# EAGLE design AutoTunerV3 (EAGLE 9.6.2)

## Sheet 1 of 4: mcu
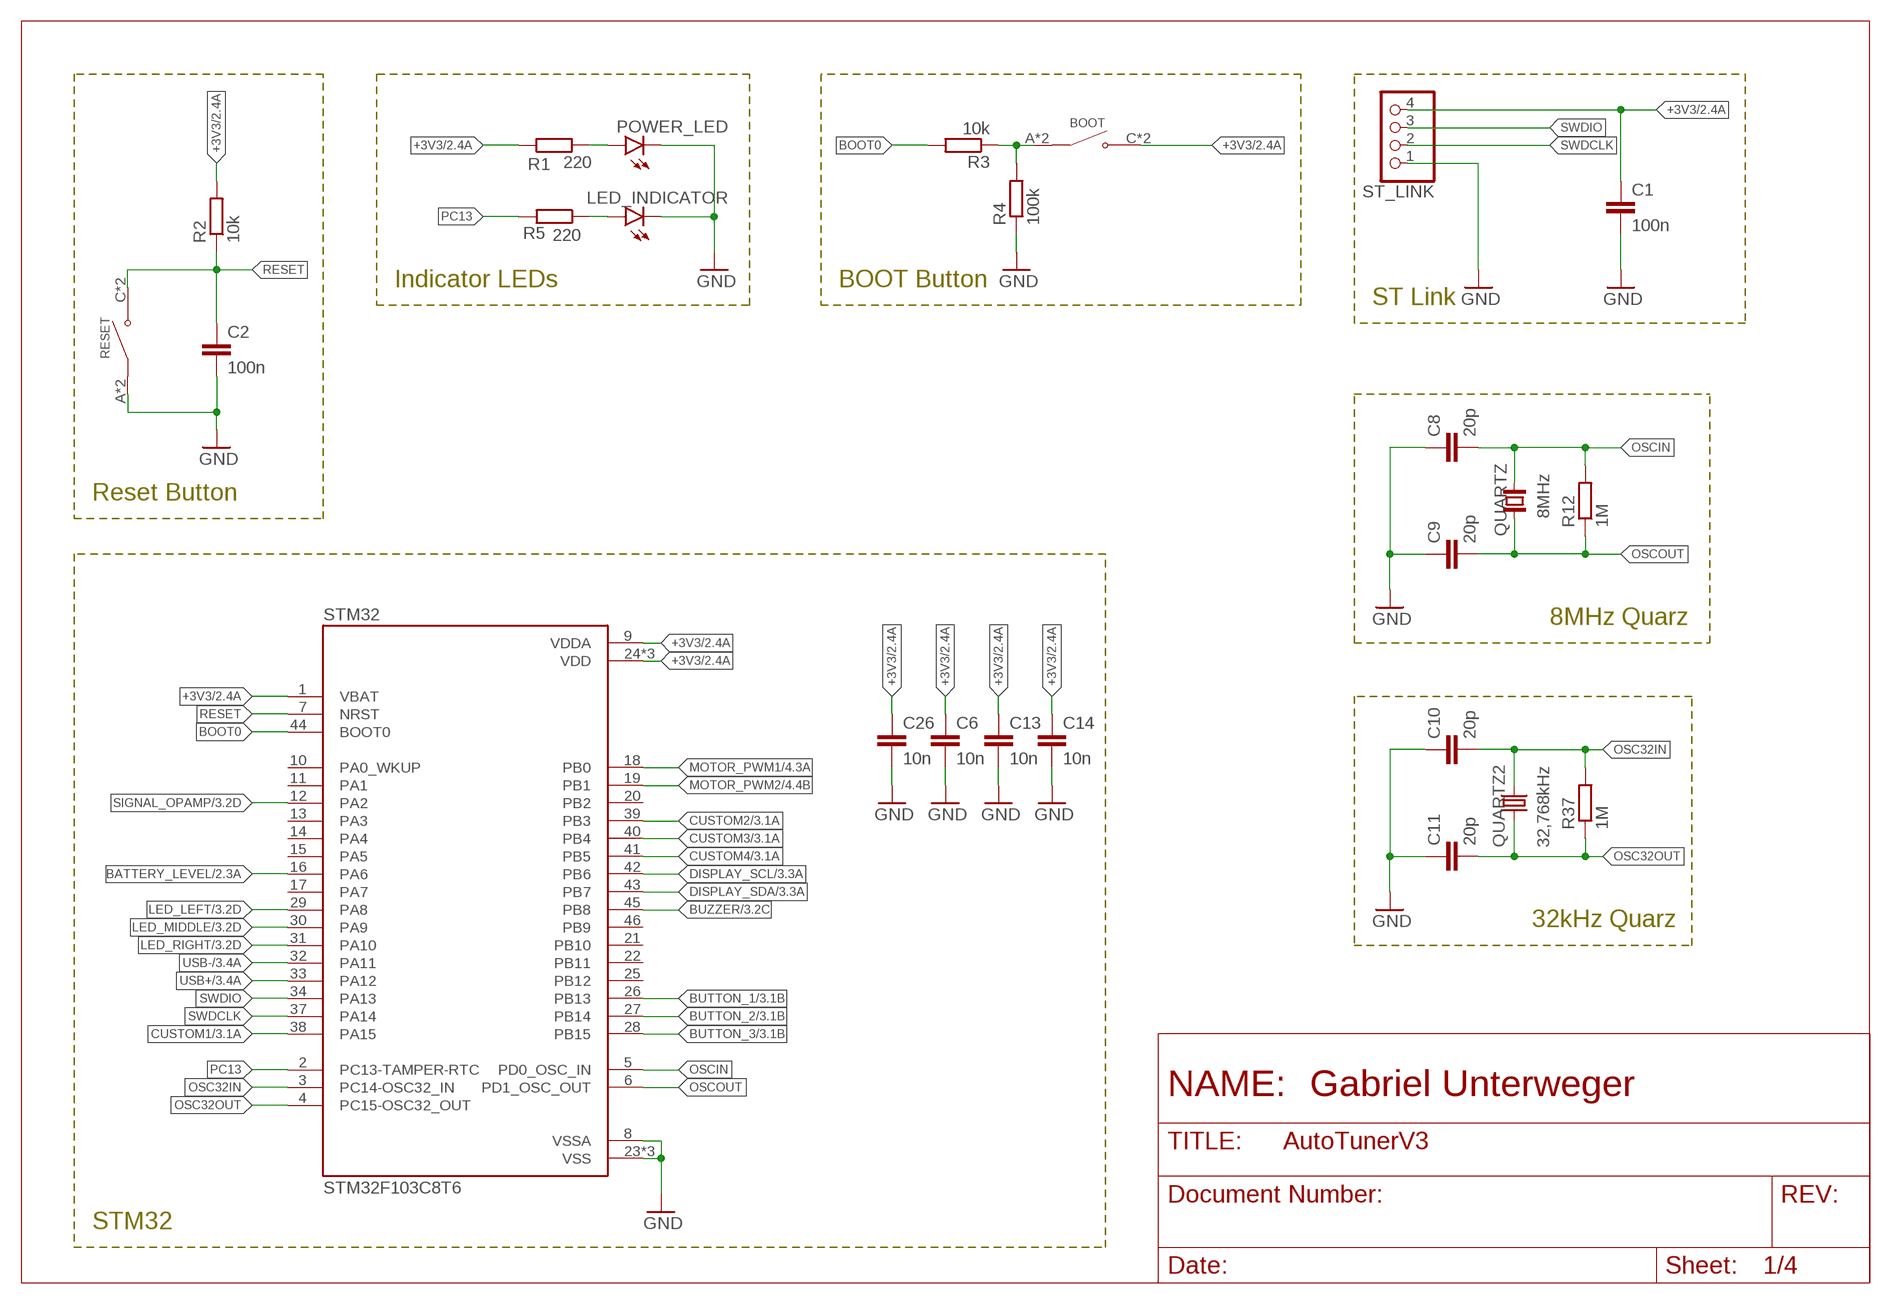
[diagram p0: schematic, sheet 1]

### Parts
BOOT  TS-1187A-B-A-B  [SW_TS-1187A-B-A-B]
C1  100n  C-EUC0805  [C0805]
C2  100n  C-EUC0805  [C0805]
C6  10n  C-EUC0805  [C0805]
C8  20p  C-EUC0805  [C0805]
C9  20p  C-EUC0805  [C0805]
C10  20p  C-EUC0805  [C0805]
C11  20p  C-EUC0805  [C0805]
C13  10n  C-EUC0805  [C0805]
C14  10n  C-EUC0805  [C0805]
C26  10n  C-EUC0805  [C0805]
LED_INDICATOR  LEDCHIPLED_0805  [CHIPLED_0805]
POWER_LED  LEDCHIPLED_0805  [CHIPLED_0805]
QUARTZ  8MHz  CRYSTAL_NX5032GA  [CRYSTAL_2-SMD-5X3]
QUARTZ2  32,768kHz  KX-327-NHF  [3.2X1.5]
R1  220  R-EU_R0805  [R0805]
R2  10k  R-EU_R0805  [R0805]
R3  10k  R-EU_R0805  [R0805]
R4  100k  R-EU_R0805  [R0805]
R5  220  R-EU_R0805  [R0805]
R12  1M  R-EU_R0805  [R0805]
R37  1M  R-EU_R0805  [R0805]
RESET  TS-1187A-B-A-B  [SW_TS-1187A-B-A-B]
ST_LINK  PINHD-1X4/90  [1X04/90]
STM32  STM32F103C8T6  [QFP50P900X900X160-48N]

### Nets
+3V3: BOOT.C(NO) BOOT.D(NO) C1.1 C6.1 C13.1 C14.1 C26.1 R1.1 R2.2 ST_LINK.4 STM32.1(VBAT) STM32.9(VDDA) STM32.24(VDD) STM32.36(VDD) STM32.48(VDD) ; also sheet 2,3,4
BATTERY_LEVEL: STM32.16(PA6) ; also sheet 2
BOOT0: R3.2 STM32.44(BOOT0)
BUTTON_1: STM32.26(PB13) ; also sheet 3
BUTTON_2: STM32.27(PB14) ; also sheet 3
BUTTON_3: STM32.28(PB15) ; also sheet 3
BUZZER: STM32.45(PB8) ; also sheet 3
CUSTOM1: STM32.38(PA15) ; also sheet 3
CUSTOM2: STM32.39(PB3) ; also sheet 3
CUSTOM3: STM32.40(PB4) ; also sheet 3
CUSTOM4: STM32.41(PB5) ; also sheet 3
DISPLAY_SCL: STM32.42(PB6) ; also sheet 3
DISPLAY_SDA: STM32.43(PB7) ; also sheet 3
GND: C1.2 C2.2 C6.2 C8.1 C9.1 C10.1 C11.1 C13.2 C14.2 C26.2 LED_INDICATOR.C POWER_LED.C R4.1 RESET.A(COM) RESET.B(COM) ST_LINK.1 STM32.8(VSSA) STM32.23(VSS) STM32.35(VSS) STM32.47(VSS) ; also sheet 2,3,4
LED_LEFT: STM32.29(PA8) ; also sheet 3
LED_MIDDLE: STM32.30(PA9) ; also sheet 3
LED_RIGHT: STM32.31(PA10) ; also sheet 3
MOTOR_PWM1: STM32.18(PB0) ; also sheet 4
MOTOR_PWM2: STM32.19(PB1) ; also sheet 4
N$1: POWER_LED.A R1.2
N$2: LED_INDICATOR.A R5.1
N$5: BOOT.A(COM) BOOT.B(COM) R3.1 R4.2
OSC32IN: C10.2 QUARTZ2.2 R37.2 STM32.3(PC14-OSC32_IN)
OSC32OUT: C11.2 QUARTZ2.1 R37.1 STM32.4(PC15-OSC32_OUT)
OSCIN: C8.2 QUARTZ.2 R12.2 STM32.5(PD0_OSC_IN)
OSCOUT: C9.2 QUARTZ.1 R12.1 STM32.6(PD1_OSC_OUT)
PC13: R5.2 STM32.2(PC13-TAMPER-RTC)
RESET: C2.1 R2.1 RESET.C(NO) RESET.D(NO) STM32.7(NRST)
SIGNAL_OPAMP: STM32.12(PA2) ; also sheet 3,4
SWDCLK: ST_LINK.2 STM32.37(PA14)
SWDIO: ST_LINK.3 STM32.34(PA13)
USB+: STM32.33(PA12) ; also sheet 3
USB-: STM32.32(PA11) ; also sheet 3
Unconnected: STM32.10(PA0_WKUP) STM32.11(PA1) STM32.13(PA3) STM32.14(PA4) STM32.15(PA5) STM32.17(PA7) STM32.20(PB2) STM32.21(PB10) STM32.22(PB11) STM32.25(PB12) STM32.46(PB9)

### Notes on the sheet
- Indicator LEDs | BOOT Button
- ST Link
- Reset Button
- 8MHz Quarz
- 32kHz Quarz
- STM32

## Sheet 2 of 4: battery / voltage converter
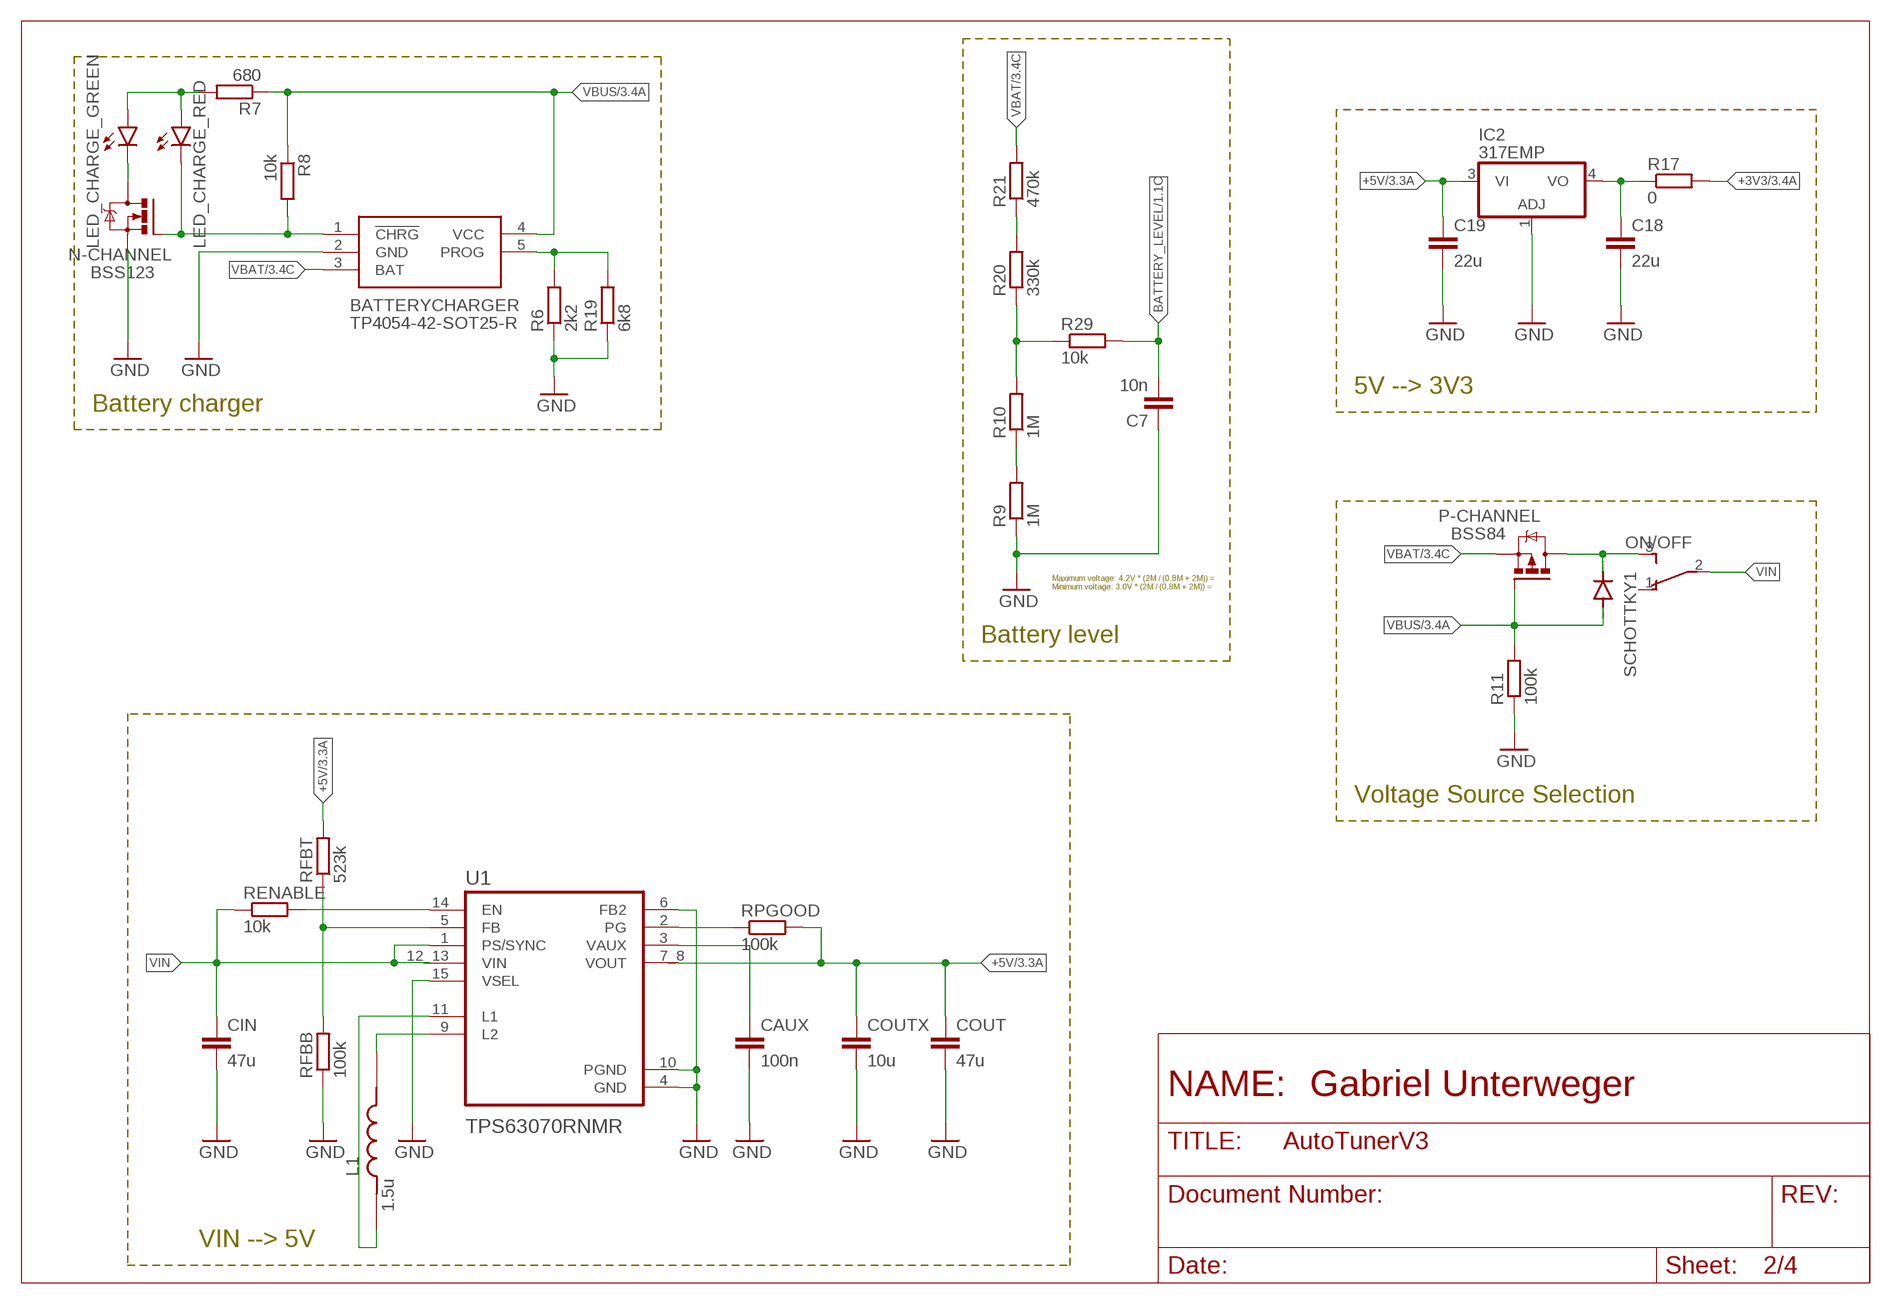
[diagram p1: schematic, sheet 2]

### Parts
BATTERYCHARGER  TP4054-42-SOT25-R  [SOT95P280X100-5N]
C7  10n  C-EUC0805  [C0805]
C18  22u  C-EUC1206  [C1206]
C19  22u  C-EUC1206  [C1206]
CAUX  100n  C-EUC0402  [C0402]
CIN  47u  C-EUC1206  [C1206]
COUT  47u  C-EUC1206  [C1206]
COUTX  10u  C-EUC0603  [C0603]
IC2  317EMP  [SOT223]
L1  1.5u  XFL4020-152MEC  [IND_XFL4020-152MEC]
LED_CHARGE_GREEN  LEDCHIPLED_0805  [CHIPLED_0805]
LED_CHARGE_RED  LEDCHIPLED_0805  [CHIPLED_0805]
N-CHANNEL  BSS123  NMOSFET_BSS123_SOT23-GSD  [SOT23]
ON/OFF  TL36PO  [TL3XPO]
P-CHANNEL  BSS84  PMOSFET_BSS84_SOT23-GSD  [SOT23]
R6  2k2  R-EU_R0805  [R0805]
R7  680  R-EU_R0805  [R0805]
R8  10k  R-EU_R0805  [R0805]
R9  1M  R-EU_R0805  [R0805]
R10  1M  R-EU_R0805  [R0805]
R11  100k  R-EU_R0805  [R0805]
R17  0  R-EU_R0805  [R0805]
R19  6k8  R-EU_R0805  [R0805]
R20  330k  R-EU_R0805  [R0805]
R21  470k  R-EU_R0805  [R0805]
R29  10k  R-EU_R0805  [R0805]
RENABLE  10k  R-EU_R0805  [R0805]
RFBB  100k  R-EU_R0805  [R0805]
RFBT  523k  R-EU_R0805  [R0805]
RPGOOD  100k  R-EU_R0805  [R0805]
SCHOTTKY1  DIODE-SOD323-R  [SOD323-R]
U1  TPS63070RNMR  [VREG_TPS63070RNMR]

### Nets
+3V3: R17.2 ; also sheet 1,3,4
+5V: C19.1 COUT.1 COUTX.1 IC2.3(VI) RFBT.2 RPGOOD.2 U1.7_8(VOUT) ; also sheet 3
BATTERY_LEVEL: C7.2 R29.2 ; also sheet 1
GND: BATTERYCHARGER.2(GND) C7.1 C18.2 C19.2 CAUX.2 CIN.2 COUT.2 COUTX.2 IC2.1(ADJ) N-CHANNEL.2(S) R6.1 R9.1 R11.1 R19.1 RFBB.1 U1.4(GND) U1.6(FB2) U1.10(PGND) U1.15(VSEL) ; also sheet 1,3,4
L1: L1.1 U1.11(L1)
L2: L1.2 U1.9(L2)
N$3: ON/OFF.3(S) P-CHANNEL.3(D) SCHOTTKY1.C
N$4: R9.2 R10.1
N$8: BATTERYCHARGER.5(PROG) R6.2 R19.2
N$9: BATTERYCHARGER.1(!CHRG) LED_CHARGE_RED.C N-CHANNEL.1(G) R8.2
N$11: LED_CHARGE_GREEN.A LED_CHARGE_RED.A R7.2
N$12: LED_CHARGE_GREEN.C N-CHANNEL.3(D)
N$13: C18.1 IC2.4(VO) R17.1
N$46: R20.2 R21.1
N$47: R10.2 R20.1 R29.1
N$60: CAUX.1 U1.3(VAUX)
N$61: RPGOOD.1 U1.2(PG)
N$62: RFBB.2 RFBT.1 U1.5(FB)
N$64: RENABLE.2 U1.14(EN)
VBAT: BATTERYCHARGER.3(BAT) P-CHANNEL.2(S) R21.2 ; also sheet 3,4
VBUS: BATTERYCHARGER.4(VCC) P-CHANNEL.1(G) R7.1 R8.1 R11.2 SCHOTTKY1.A ; also sheet 3
VIN: CIN.1 ON/OFF.2(P) RENABLE.1 U1.1(PS/SYNC) U1.12_13(VIN)
Unconnected: ON/OFF.1(O)

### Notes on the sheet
- 5V --> 3V3
- Battery charger
- Maximum voltage: 4.2V * (2M / (0.8M + 2M)) =
  Minimum voltage: 3.0V * (2M / (0.8M + 2M)) =
- Battery level
- Voltage Source Selection
- VIN --> 5V

## Sheet 3 of 4: I/O
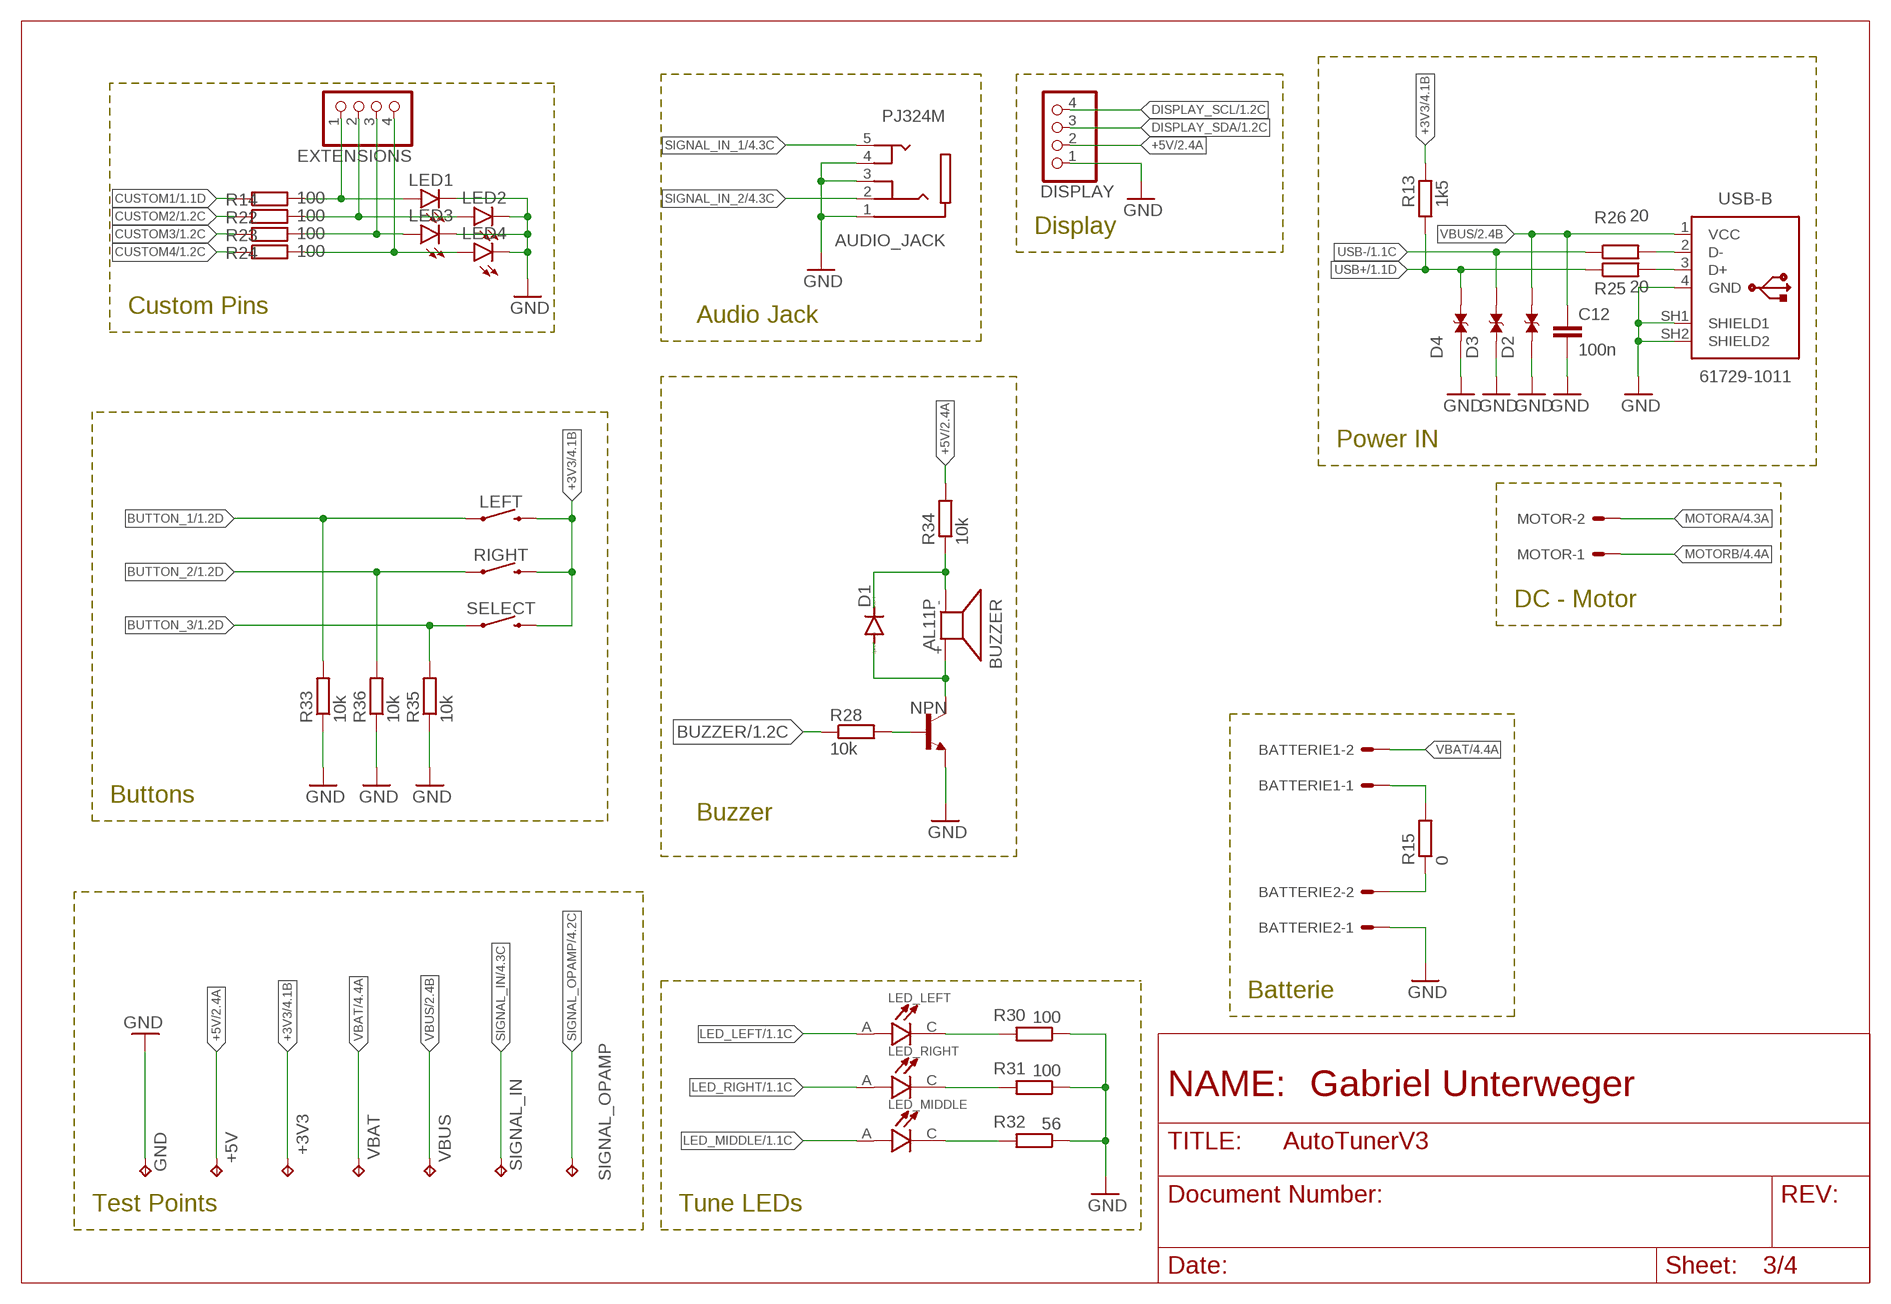
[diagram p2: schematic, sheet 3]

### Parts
+3V3  TPB1,27  [B1,27]
+5V  TPB1,27  [B1,27]
AUDIO_JACK  PJ324M  [WENZHOU_PJ324M]
BATTERIE1  22-27-2021-02  [6410-02]
BATTERIE2  22-27-2021-02  [6410-02]
BUZZER  AL11P  [AL11P]
C12  100n  C-EUC0805  [C0805]
D1  DIODE-SOD323-R  [SOD323-R]
D2  TESD5V0L1UC_RJG  [DIO_TESD5V0L1UC_RJG]
D3  TESD5V0L1UC_RJG  [DIO_TESD5V0L1UC_RJG]
D4  TESD5V0L1UC_RJG  [DIO_TESD5V0L1UC_RJG]
DISPLAY  PINHD-1X4  [1X04]
EXTENSIONS  PINHD-1X4/90  [1X04/90]
GND  TPB1,27  [B1,27]
LED1  LEDCHIP-LED0805  [CHIP-LED0805]
LED2  LEDCHIP-LED0805  [CHIP-LED0805]
LED3  LEDCHIP-LED0805  [CHIP-LED0805]
LED4  LEDCHIP-LED0805  [CHIP-LED0805]
LED_LEFT  L-53GD  [LEDRD254W50D500H1060]
LED_MIDDLE  L-53GD  [LEDRD254W50D500H1060]
LED_RIGHT  L-53GD  [LEDRD254W50D500H1060]
LEFT  MOMENTARY-SWITCH-SPST-PTH-12MM  [TACTILE_SWITCH_PTH_12MM]
MOTOR  22-27-2021-02  [6410-02]
NPN  -NPN-SOT23-EBC  [SOT23-EBC]
R13  1k5  R-EU_R0805  [R0805]
R14  100  R-EU_R0805  [R0805]
R15  0  R-EU_R0805  [R0805]
R22  100  R-EU_R0805  [R0805]
R23  100  R-EU_R0805  [R0805]
R24  100  R-EU_R0805  [R0805]
R25  20  R-EU_R0805  [R0805]
R26  20  R-EU_R0805  [R0805]
R28  10k  R-EU_R0805  [R0805]
R30  100  R-EU_R0805  [R0805]
R31  100  R-EU_R0805  [R0805]
R32  56  R-EU_R0805  [R0805]
R33  10k  R-EU_R0805  [R0805]
R34  10k  R-EU_R0805  [R0805]
R35  10k  R-EU_R0805  [R0805]
R36  10k  R-EU_R0805  [R0805]
RIGHT  MOMENTARY-SWITCH-SPST-PTH-12MM  [TACTILE_SWITCH_PTH_12MM]
SELECT  MOMENTARY-SWITCH-SPST-PTH-12MM  [TACTILE_SWITCH_PTH_12MM]
SIGNAL_IN  TPB1,27  [B1,27]
SIGNAL_OPAMP  TPB1,27  [B1,27]
USB-B  61729-1011  [61729-1011BLF]
VBAT  TPB1,27  [B1,27]
VBUS  TPB1,27  [B1,27]

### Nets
+3V3: +3V3.TP LEFT.3 R13.2 RIGHT.3 SELECT.3 ; also sheet 1,2,4
+5V: +5V.TP DISPLAY.2 R34.2 ; also sheet 2
BUTTON_1: LEFT.1 R33.2 ; also sheet 1
BUTTON_2: R36.2 RIGHT.1 ; also sheet 1
BUTTON_3: R35.2 SELECT.1 ; also sheet 1
BUZZER: R28.1 ; also sheet 1
CUSTOM1: R14.1 ; also sheet 1
CUSTOM2: R22.1 ; also sheet 1
CUSTOM3: R23.1 ; also sheet 1
CUSTOM4: R24.1 ; also sheet 1
DISPLAY_SCL: DISPLAY.4 ; also sheet 1
DISPLAY_SDA: DISPLAY.3 ; also sheet 1
GND: AUDIO_JACK.1(SLEEVE) AUDIO_JACK.3(RING_2) AUDIO_JACK.4(TIP_1) BATTERIE2.1 C12.2 D2.1 D3.1 D4.1 DISPLAY.1 GND.TP LED1.C LED2.C LED3.C LED4.C NPN.E R30.1 R31.1 R32.1 R33.1 R35.1 R36.1 USB-B.4(GND) USB-B.SH1(SHIELD1) USB-B.SH2(SHIELD2) ; also sheet 1,2,4
LED_LEFT: LED_LEFT.A ; also sheet 1
LED_MIDDLE: LED_MIDDLE.A ; also sheet 1
LED_RIGHT: LED_RIGHT.A ; also sheet 1
MOTORA: MOTOR.2 ; also sheet 4
MOTORB: MOTOR.1 ; also sheet 4
N$19: LED_LEFT.C R30.2
N$20: LED_RIGHT.C R31.2
N$23: LED_MIDDLE.C R32.2
N$29: R25.2 USB-B.3(D+)
N$30: R26.2 USB-B.2(D-)
N$39: EXTENSIONS.1 LED1.A R14.2
N$48: EXTENSIONS.2 LED2.A R22.2
N$49: EXTENSIONS.3 LED3.A R23.2
N$50: EXTENSIONS.4 LED4.A R24.2
N$51: BATTERIE2.2 R15.1
N$53: BATTERIE1.1 R15.2
N$54: BUZZER.+ D1.A NPN.C
N$55: BUZZER.- D1.C R34.1
N$56: NPN.B R28.2
SIGNAL_IN: SIGNAL_IN.TP ; also sheet 4
SIGNAL_IN_1: AUDIO_JACK.5(TIP_2) ; also sheet 4
SIGNAL_IN_2: AUDIO_JACK.2(RING_1) ; also sheet 4
SIGNAL_OPAMP: SIGNAL_OPAMP.TP ; also sheet 1,4
USB+: D4.2 R13.1 R25.1 ; also sheet 1
USB-: D3.2 R26.1 ; also sheet 1
VBAT: BATTERIE1.2 VBAT.TP ; also sheet 2,4
VBUS: C12.1 D2.2 USB-B.1(VCC) VBUS.TP ; also sheet 2

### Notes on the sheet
- Display
- Custom Pins
- Audio Jack
- Power IN
- DC - Motor
- Buttons
- Buzzer
- Batterie
- Test Points | Tune LEDs

## Sheet 4 of 4: Motor Steuerung / Signal Verarbeitung
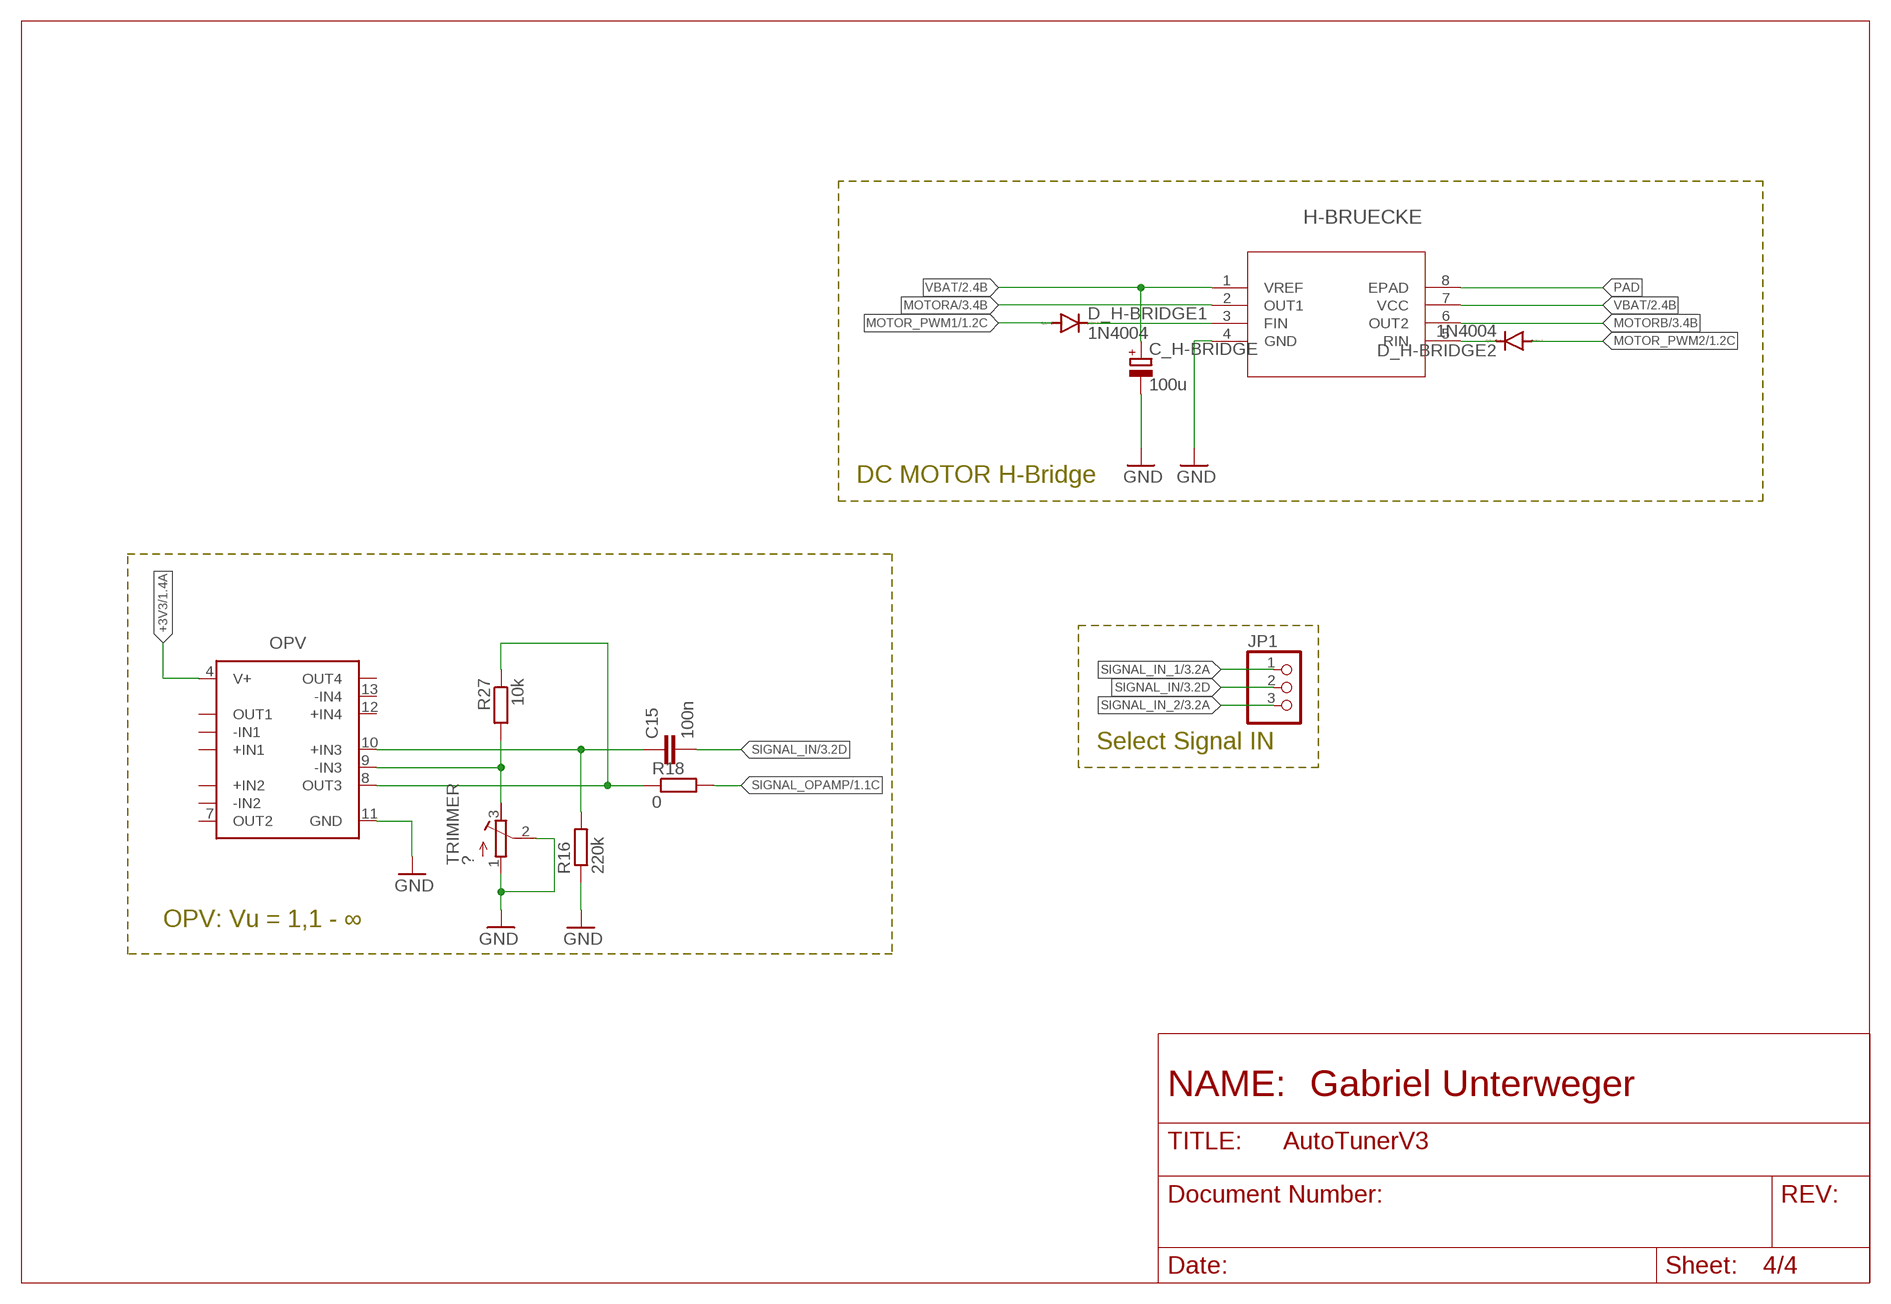
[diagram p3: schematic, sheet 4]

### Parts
C15  100n  C-EUC0805  [C0805]
C_H-BRIDGE  100u  CPOL-EUE2,5-6E  [E2,5-6E]
D_H-BRIDGE1  1N4004  [DO41-10]
D_H-BRIDGE2  1N4004  [DO41-10]
H-BRUECKE  BD6222HFP-TRHRP7_ROM-M  [HRP7_ROM-M]
JP1  PINHD-1X3  [1X03]
OPV  LM324_SOIC  [SOIC127P600X175-14N]
R16  220k  R-EU_R0805  [R0805]
R18  0  R-EU_R0805  [R0805]
R27  10k  R-EU_R0805  [R0805]
TRIMMER  ?  R-TRIMM3339P  [RTRIM3339P]

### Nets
+3V3: OPV.4(V+) ; also sheet 1,2,3
GND: C_H-BRIDGE.- H-BRUECKE.4(GND) OPV.11(GND) R16.1 TRIMMER.1(A) TRIMMER.2(S) ; also sheet 1,2,3
MOTOR_PWM1: D_H-BRIDGE1.A ; also sheet 1
MOTOR_PWM2: D_H-BRIDGE2.A ; also sheet 1
MOTORA: H-BRUECKE.2(OUT1) ; also sheet 3
MOTORB: H-BRUECKE.6(OUT2) ; also sheet 3
N$6: D_H-BRIDGE1.C H-BRUECKE.3(FIN)
N$7: OPV.8(OUT3) R18.1 R27.1
N$14: D_H-BRIDGE2.C H-BRUECKE.5(RIN)
N$16: OPV.9(-IN3) R27.2 TRIMMER.3(E)
N$52: C15.1 OPV.10(+IN3) R16.2
PAD: H-BRUECKE.8(EPAD)
SIGNAL_IN: C15.2 JP1.2 ; also sheet 3
SIGNAL_IN_1: JP1.1 ; also sheet 3
SIGNAL_IN_2: JP1.3 ; also sheet 3
SIGNAL_OPAMP: R18.2 ; also sheet 1,3
VBAT: C_H-BRIDGE.+ H-BRUECKE.1(VREF) H-BRUECKE.7(VCC) ; also sheet 2,3
Unconnected: OPV.1(OUT1) OPV.2(-IN1) OPV.3(+IN1) OPV.5(+IN2) OPV.6(-IN2) OPV.7(OUT2) OPV.12(+IN4) OPV.13(-IN4) OPV.14(OUT4)

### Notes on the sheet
- DC MOTOR H-Bridge
- Select Signal IN
- OPV: Vu = 1,1 - ∞

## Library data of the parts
+3V3 +5V GND SIGNAL_IN SIGNAL_OPAMP VBAT VBUS = testpad:TP: Test pad
AUDIO_JACK = PJ324M:PJ324M: Headphone Stereo jack/Audio connector Check availability; AVAILABILITY: Not in stock; CHECK_PRICES: https://www.snapeda.com/parts/PJ324M/Wenzhou+QingPu+Electronics+Co.Ltd/view-part/?ref=eda; DESCRIPTION: Headphone Stereo jack/Audio connector; MF: Wenzhou QingPu Electronics Co.Ltd; MP: PJ324M; PACKAGE: Package; PRICE: None; SNAPEDA_LINK: https://www.snapeda.com/parts/PJ324M/Wenzhou+QingPu+Electronics+Co.Ltd/view-part/?ref=snap
BATTERIE1 BATTERIE2 MOTOR = con-molex:22-?-02: CONNECTOR; MF: MOLEX; OC_FARNELL: unknown; OC_NEWARK: unknown
BATTERYCHARGER = TP4054-42-SOT25-R:TP4054-42-SOT25-R: Standalone Linear Li-ion Battery Charger with Thermal Regulation, SOT-23-5 Source: Datasheet; DESCRIPTION: Standalone Linear Li-ion Battery Charger with Thermal Regulation, SOT-23-5; HEIGHT: 1mm; LCSC_PART: C32574; MANUFACTURER_NAME: TOP POWER; MANUFACTURER_PART_NUMBER: TP4054-42-SOT25-R
BOOT RESET = TS-1187A-B-A-B:TS-1187A-B-A-B: SPST 50mA @ 12VDC Top Actuated Round Button 160gf SMD Tactile Switches RoHS Check availability; AVAILABILITY: Not in stock; DESCRIPTION: TS-1187A-B-A-B XKB Connectivity; LCSC_PART: C318884; MF: XKB Industrial Precision; MP: TS-1187A-B-A-B; PACKAGE: Package; PRICE: None
BUZZER = buzzer:AL11P: SPEAKER; OC_FARNELL: unknown; OC_NEWARK: unknown
C1 C2 C6-C15 C26 = rcl:C-EU: CAPACITOR, European symbol; SPICEPREFIX: C
C18 C19 = rcl:C-EU: CAPACITOR, European symbol; LCSC_PART: C12891; SPICEPREFIX: C
C_H-BRIDGE = rcl:CPOL-EU: POLARIZED CAPACITOR, European symbol; SPICEPREFIX: C
CAUX = rcl:C-EU: CAPACITOR, European symbol; LCSC_PART: C1525; SPICEPREFIX: C
CIN COUT = rcl:C-EU: CAPACITOR, European symbol; LCSC_PART: C96123; SPICEPREFIX: C
COUTX = rcl:C-EU: CAPACITOR, European symbol; LCSC_PART: C19702; SPICEPREFIX: C
D1 = diode:DIODE-: DIODE; LCSC_PART: C2128
D2-D4 = TESD5V0L1UC_RJG:TESD5V0L1UC_RJG: Check availability; AVAILABILITY: In Stock; CHECK_PRICES: https://www.snapeda.com/parts/TESD5V0L1UC%20RJG/Taiwan+Semiconductor/view-part/?ref=eda; DESCRIPTION: DFN1006L, 5V, 100W, 2pF, ESD Protection Diode & Array; LCSC_PART: C7420372; MF: Taiwan Semiconductor Corporation; MP: TESD5V0L1UC RJG; PACKAGE: DFN1006L Taiwan Semiconductor; PRICE: None; PURCHASE-URL: https://www.snapeda.com/api/url_track_click_mouser/?unipart_id=3789592&manufacturer=Taiwan Semiconductor Corporation&part_name=TESD5V0L1UC RJG&search_term=protection diode; SNAPEDA_LINK: https://www.snapeda.com/parts/TESD5V0L1UC%20RJG/Taiwan+Semiconductor/view-part/?ref=snap
D_H-BRIDGE1 D_H-BRIDGE2 = diode:1N4004: DIODE
DISPLAY EXTENSIONS ST_LINK = pinhead:PINHD-1X4: PIN HEADER
H-BRUECKE = H-Brücke_BD622HFP-TR02:BD6222HFP-TR; COPYRIGHT: Copyright (C) 2022 Ultra Librarian. All rights reserved.; MANUFACTURER_PART_NUMBER: BD6222HFP-TR; MFR_NAME: ROHM Semiconductor
IC2 = linear:*317: Positive VOLTAGE REGULATOR; LCSC_PART: C6186
JP1 = pinhead:PINHD-1X3: PIN HEADER
L1 = XFL4020-152MEC:XFL4020-152MEC: Power inductor, shielded, 20% tol, SMT, RoHS, halogen free Check availability; AVAILABILITY: In Stock; CHECK_PRICES: https://www.snapeda.com/parts/XFL4020-152MEC/Coilcraft/view-part/?ref=eda; DESCRIPTION: Inductor Power Shielded Wirewound 1.5uH 20% 100KHz 9.1A 15.8mOhm DCR 1515 Automotive Embossed Plastic T/R; LCSC_PART: C3033018; MF: Coilcraft; MP: XFL4020-152MEC; PACKAGE: None; PRICE: None; PURCHASE-URL: https://www.snapeda.com/api/url_track_click_mouser/?unipart_id=583942&manufacturer=Coilcraft&part_name=XFL4020-152MEC&search_term=xfl4020-152mec; SNAPEDA_LINK: https://www.snapeda.com/parts/XFL4020-152MEC/Coilcraft/view-part/?ref=snap
LED1-LED4 LED_CHARGE_GREEN POWER_LED = led:LED: LED; LCSC_PART: C2297
LED_CHARGE_RED = led:LED: LED; LCSC_PART: C84256
LED_INDICATOR = led:LED: LED; LCSC_PART: C2296
LED_LEFT LED_MIDDLE LED_RIGHT = L-53GD:L-53GD: LED; 5mm; green; 5-32mcd; 60°; Front: convex Check availability; AVAILABILITY: In Stock; CHECK_PRICES: https://www.snapeda.com/parts/L-53GD/Kingbright/view-part/?ref=eda; DESCRIPTION: LED; 5mm; green; 5-32mcd; 60°; Front: convex; MF: Kingbright; MP: L-53GD; PACKAGE: CDIP-28 Kingbright; PRICE: None; PURCHASE-URL: https://www.snapeda.com/api/url_track_click_mouser/?unipart_id=525636&manufacturer=Kingbright&part_name=L-53GD&search_term=led, 5mm; SNAPEDA_LINK: https://www.snapeda.com/parts/L-53GD/Kingbright/view-part/?ref=snap
LEFT RIGHT SELECT = SparkFun-Switches:MOMENTARY-SWITCH-SPST: Momentary Switch (Pushbutton) - SPST; PROD_ID: SWCH-09185; SF_SKU: COM-09190
N-CHANNEL = Transistor:NMOSFET_: N-Channel MOSFET - Popular parts; CATEGORY: Transistor; DESCRIPTION: MOSFET N-CH 100V 0.17A SOT-23; DRAIN_CURRENT: 170mA; LCSC_PART: C20917; MANUFACTURER: ON Semiconductor; MPN: BSS123L; OPERATING_TEMP: -55°C ~ 150°C; PART_STATUS: Active; ROHS_COMPLIANT: Yes; SUB-CATEGORY: MOSFET; THERMALLOSS: 360mW; TYPE: N-Channel
NPN = transistor:*-NPN-: NPN Transistror BF959 corrected 2008.03.06; LCSC_PART: C364312
ON/OFF = switch:TL36PO: TINY SWITCH ON - ON Source: http://www2.produktinfo.conrad.com/datenblaetter/700000-724999/705152-da-01-de-Subminiaturschalter_TL_36YO.pdf
OPV = IC_Linear:LM324: Quad-Operational Amplifiers Reference Datasheet; CATEGORY: Operational Amplifiers; DESCRIPTION: Quad-Operational Amplifiers; LCSC_PART: C71035; MANUFACTURER: Generic; MPN: Generic; SERIES: LM324; SUB-CATEGORY: Amplifier ICs; TYPE: Op Amps - Operational Amplifiers
P-CHANNEL = Transistor:PMOSFET_: P-Channel MOSFET - Popular parts; CATEGORY: Transistor; DESCRIPTION: MOSFET P-CH 50V 130MA SOT-23; DRAIN_CURRENT: 130mA; LCSC_PARTS: C10487; MANUFACTURER: ON Semiconductor; MPN: BSS84; OPERATING_TEMP: -55°C ~ 150°C; PART_STATUS: Active; ROHS_COMPLIANT: Yes; SUB-CATEGORY: MOSFET; THERMALLOSS: 360mW; TYPE: P-Channel
QUARTZ = 52101-101-REV-A_v16:CRYSTAL_NX5032GA: CRYSTAL; LCSC_PART: C115962
QUARTZ2 = crystal-geyer_V1_0:KX-327; LCSC_PART: C32346
R1 = rcl:R-EU_: RESISTOR, European symbol; LCSC_PART: C17557; SPICEPREFIX: R
R2-R4 R6-R37 RENABLE RFBB RFBT RPGOOD = rcl:R-EU_: RESISTOR, European symbol; SPICEPREFIX: R
R5 = rcl:R-EU_: RESISTOR, European symbol; LCSC_PART: C17802; SPICEPREFIX: R
SCHOTTKY1 = diode:DIODE-: DIODE; LCSC_PART: C191023
STM32 = STM32F103C8T6:STM32F103C8T6: Mainstream Performance line, ARM Cortex-M3 MCU with 64 Kbytes Flash, 72 MHz CPU, motor control, USB and CAN Check availability; AVAILABILITY: In Stock; CHECK_PRICES: https://www.snapeda.com/parts/STM32F103C8T6/STMicroelectronics/view-part/?ref=eda; DESCRIPTION: ARM® Cortex®-M3 STM32F1 Microcontroller IC 32-Bit 72MHz 64KB (64K x 8) FLASH 48-LQFP (7x7); LCSC_PART: C8734; MF: STMicroelectronics; MP: STM32F103C8T6; PACKAGE: LQFP-48 STMicroelectronics; PRICE: None; PURCHASE-URL: https://www.snapeda.com/api/url_track_click_mouser/?unipart_id=52195&manufacturer=STMicroelectronics&part_name=STM32F103C8T6&search_term=stm32f103c8t6; SNAPEDA_LINK: https://www.snapeda.com/parts/STM32F103C8T6/STMicroelectronics/view-part/?ref=snap
TRIMMER = rcl:R-TRIMM: Trimm resistor; SPICEMODEL: X; SPICEPREFIXL: POT
U1 = TPS63070RNMR:TPS63070RNMR: Check availability; AVAILABILITY: In Stock; CHECK_PRICES: https://www.snapeda.com/parts/TPS63070RNMR/Texas+Instruments/view-part/?ref=eda; DESCRIPTION: Wide input voltage (2V-16V) buck-boost converter; LCSC_PART: C109322; MF: Texas Instruments; MP: TPS63070RNMR; PACKAGE: VQFN-HR-15 Texas Instruments; PRICE: None; PURCHASE-URL: https://www.snapeda.com/api/url_track_click_mouser/?unipart_id=583017&manufacturer=Texas Instruments&part_name=TPS63070RNMR&search_term=tps63070rnmr; SNAPEDA_LINK: https://www.snapeda.com/parts/TPS63070RNMR/Texas+Instruments/view-part/?ref=snap
USB-B = Connector_USB:61729-1011: USB(2.0) Type-B, RCPT, 4POS, THT-R/A Datasheet; CATEGORY: Connector; CONTACTS: 4; CURRENT_RATING: 1A; DESCRIPTION: CONN RCPT USB2.0 TYPEB 4POS R/A; GENDER: Receptacle; MANUFACTURER: Amphenol ICC (FCI); MOUNT_TYPE: R/A; MPN: 61729-1011BLF; OPERATING_TEMP: -55°C to 85°C; PART_STATUS: Active; ROHS_COMPLIANT: RoHS Compliant; SERIES: 61729; SUB-CATEGORY: USB; TYPE: USB-B

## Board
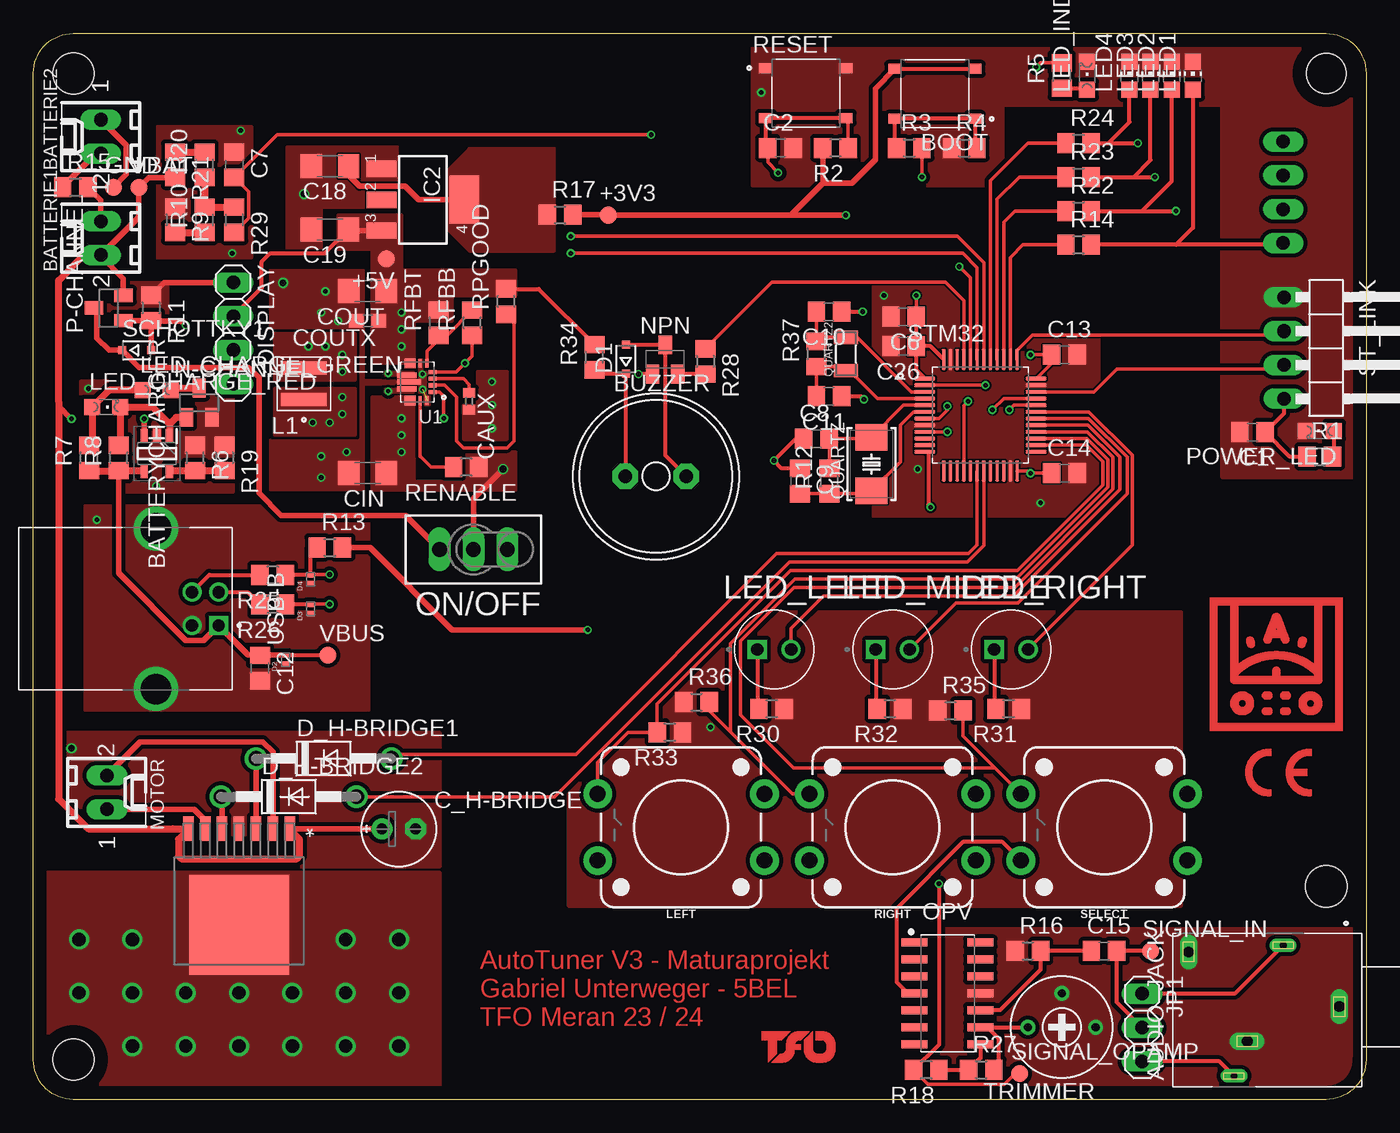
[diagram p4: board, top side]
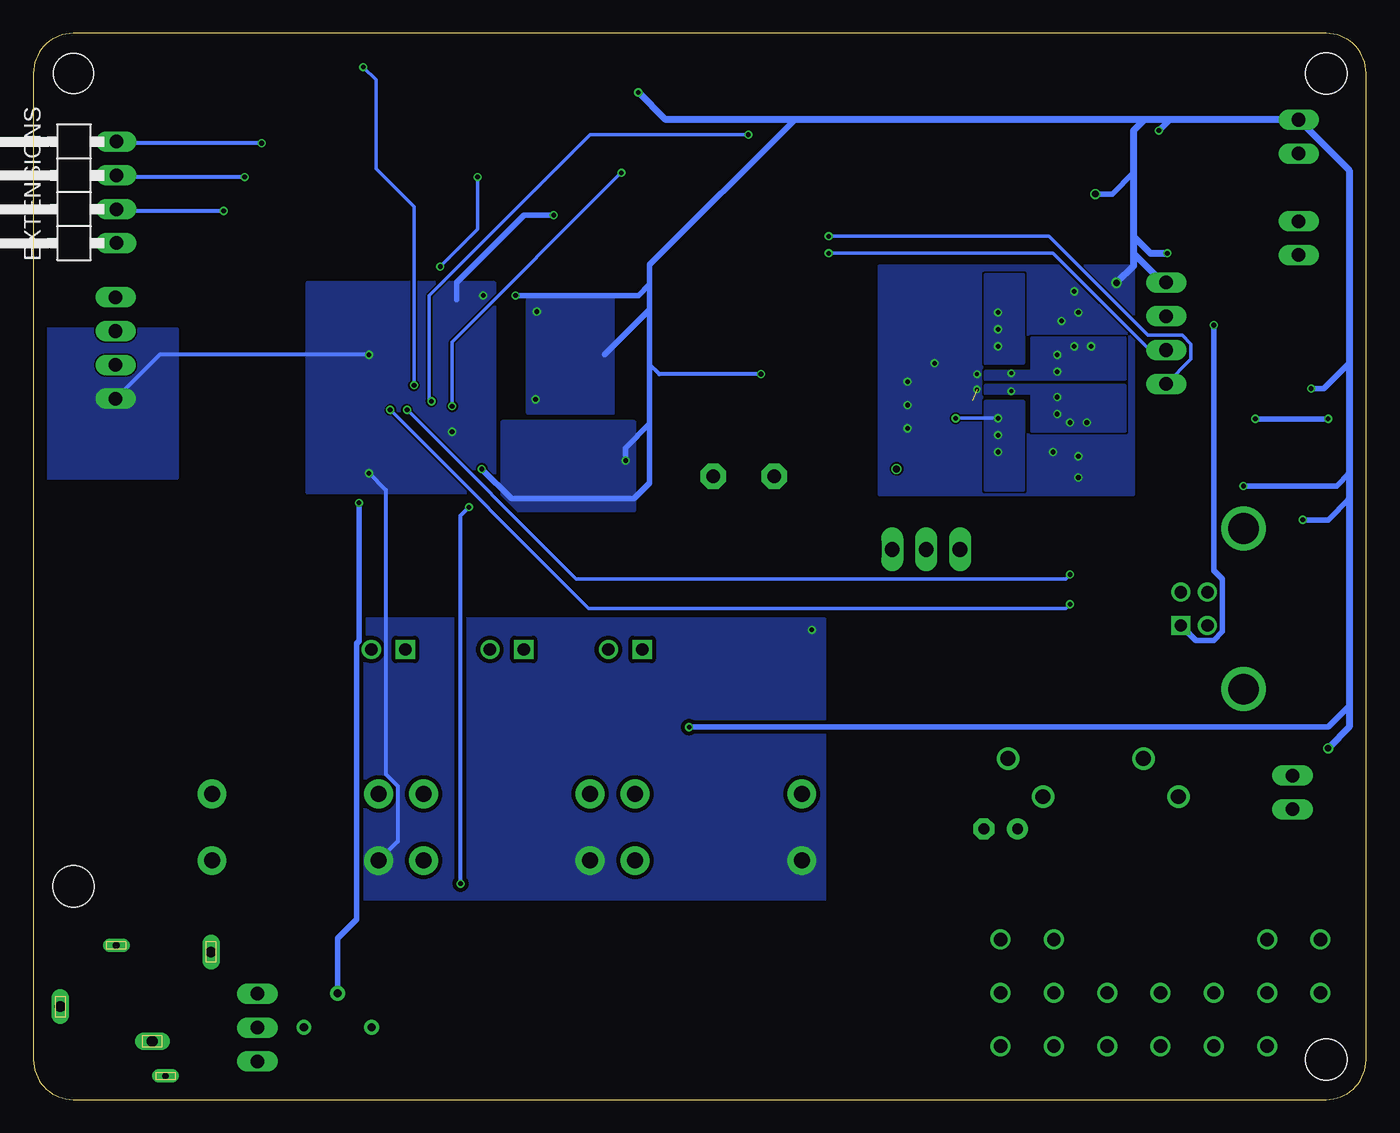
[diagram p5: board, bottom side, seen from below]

Size 100 x 80 mm. Coordinates in mm from the lower left corner, seen from the top.
Outline: 0,3 0,77 arc-90 3,80 97,80 arc-90 100,77 100,3 arc-90 97,0 3,0 arc-90 0,3
Copper layers (1*16): Top 0.035mm / dielectric 1.5mm / Bottom 0.035mm
Design rules "default *": minimum track width 6mil, minimum drill 0.3mm, track to track 5mil, track to pad 0.2mm, pad to pad 5mil, via to via 0.5mm, smd to smd 5mil, copper to edge 40mil, drill to drill 5mil, minimum pad ring 10mil, minimum via ring 0.13mm, stop-mask expansion 4mil, vias tented up to drill 0mil, thermal gap 10mil
Holes 3.1 mm at 3,77 3,3 97,16
Holes 3 mm at 97,77

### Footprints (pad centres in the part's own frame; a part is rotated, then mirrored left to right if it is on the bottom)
B1,27 = smd 1.27 x 1.27: TP 0,0
WENZHOU_PJ324M = drill 0.8 long: 1 0,5.4; 3 2.6,-1.5; 4 -4.1,-5.9 | drill 0.5 long: 2 5.2,-2.5; 5 -4.6,1.2
6410-02 = drill 1.016 long: 1 1.27,0; 2 -1.27,0
SOT95P280X100-5N = smd 1.05 x 0.55: 1 -1.3,0.95; 2 -1.3,0; 3 -1.3,-0.95; 4 1.3,-0.95; 5 1.3,0.95
SW_TS-1187A-B-A-B = smd 1 x 0.75: A -3,1.875; B 3,1.875; C -3,-1.875; D 3,-1.875
AL11P = drill 1.016 pad 1.905 octagon: + 2.286,0; - -2.286,0
C0805 = smd 1.3 x 1.5: 1 -0.95,0; 2 0.95,0
C1206 = smd 1.6 x 1.8: 1 -1.4,0; 2 1.4,0
E2,5-6E = drill 0.813 pad 1.575: + -1.27,0 | drill 0.813 pad 1.575 octagon: - 1.27,0
C0402 = smd 0.7 x 0.9: 1 -0.65,0; 2 0.65,0
C0603 = smd 1.1 x 1: 1 -0.85,0; 2 0.85,0
SOD323-R = smd 0.6 x 0.6: A 1.1,0; C -1.1,0
DIO_TESD5V0L1UC_RJG = smd 0.41 x 0.56: 1 -0.35,0; 2 0.35,0
DO41-10 = drill 1.118: A 5.08,0; C -5.08,0
1X04 = drill 1.016 long: 1 -3.81,0; 2 -1.27,0; 3 1.27,0; 4 3.81,0
1X04/90 = drill 1.016 long: 1 -3.81,-3.81; 2 -1.27,-3.81; 3 1.27,-3.81; 4 3.81,-3.81
HRP7_ROM-M = smd 0.787 x 1.854: 1 -3.81,-6.172; 2 -2.54,-6.172; 3 -1.27,-6.172; 4 0,-6.172; 5 1.27,-6.172; 6 2.54,-6.172; 7 3.81,-6.172 | smd 7.48 x 7.49: 8 0,1.051
SOT223 = smd 1.219 x 2.235: 1 -2.311,-3.099; 2 0,-3.099; 3 2.311,-3.099 | smd 3.6 x 2.2: 4 0,3.099
1X03 = drill 1.016 long: 1 -2.54,0; 2 0,0; 3 2.54,0
IND_XFL4020-152MEC = smd 0.98 x 3.4: 1 -1.185,0; 2 1.185,0
CHIP-LED0805 = smd 1.2 x 1.2: A 0,-1.05; C 0,1.05
CHIPLED_0805 = smd 1.2 x 1.2: A 0,-1.05; C 0,1.05
LEDRD254W50D500H1060 = drill 0.93 pad 1.4: A 1.27,0 | drill 0.93 pad 1.4 square: C -1.27,0
TACTILE_SWITCH_PTH_12MM = drill 1.2 pad 2.159: 1 6.25,-2.5; 2 -6.25,-2.5; 3 6.25,2.5; 4 -6.25,2.5
SOT23 = smd 1 x 1.4: 1 -0.95,-1.1; 2 0.95,-1.1; 3 0,1.1
SOT23-EBC = smd 1 x 1.4: B 0.95,-1.1; C 0,1.1; E -0.95,-1.1
TL3XPO = drill 1.1 pad 1.422 long: 1 -2.54,0; 2 0,0; 3 2.54,0
SOIC127P600X175-14N = smd 1.968 x 0.599: 1 -2.473,3.81; 2 -2.473,2.54; 3 -2.473,1.27; 4 -2.473,0; 5 -2.473,-1.27; 6 -2.473,-2.54; 7 -2.473,-3.81; 8 2.473,-3.81; 9 2.473,-2.54; 10 2.473,-1.27; 11 2.473,0; 12 2.473,1.27; 13 2.473,2.54; 14 2.473,3.81
CRYSTAL_2-SMD-5X3 = smd 2 x 2.4: 1 -2,0; 2 2,0
3.2X1.5 = smd 1 x 1.8: 1 -1.25,0; 2 1.25,0
R0805 = smd 1.3 x 1.5: 1 -0.95,0; 2 0.95,0
QFP50P900X900X160-48N = smd 1.56 x 0.28: 1 -4.18,2.75; 2 -4.18,2.25; 3 -4.18,1.75; 4 -4.18,1.25; 5 -4.18,0.75; 6 -4.18,0.25; 7 -4.18,-0.25; 8 -4.18,-0.75; 9 -4.18,-1.25; 10 -4.18,-1.75; 11 -4.18,-2.25; 12 -4.18,-2.75; 25 4.18,-2.75; 26 4.18,-2.25; 27 4.18,-1.75; 28 4.18,-1.25; 29 4.18,-0.75; 30 4.18,-0.25; 31 4.18,0.25; 32 4.18,0.75; 33 4.18,1.25; 34 4.18,1.75; 35 4.18,2.25; 36 4.18,2.75 | smd 0.28 x 1.56: 13 -2.75,-4.18; 14 -2.25,-4.18; 15 -1.75,-4.18; 16 -1.25,-4.18; 17 -0.75,-4.18; 18 -0.25,-4.18; 19 0.25,-4.18; 20 0.75,-4.18; 21 1.25,-4.18; 22 1.75,-4.18; 23 2.25,-4.18; 24 2.75,-4.18; 37 2.75,4.18; 38 2.25,4.18; 39 1.75,4.18; 40 1.25,4.18; 41 0.75,4.18; 42 0.25,4.18; 43 -0.25,4.18; 44 -0.75,4.18; 45 -1.25,4.18; 46 -1.75,4.18; 47 -2.25,4.18; 48 -2.75,4.18
RTRIM3339P = drill 0.61: 1 -2.54,0; 2 0,-2.54; 3 2.54,0
VREG_TPS63070RNMR = smd 0.6 x 0.25: 1 -1.15,0.75; 2 -1.15,0.25; 3 -1.15,-0.25; 4 -1.15,-0.75 | smd 0.25 x 0.6: 5 -0.725,-1.4; 6 -0.225,-1.4; 14 -0.225,1.4; 15 -0.725,1.4 | smd 0.85 x 0.7: 7_8 0.525,-1.4; 12_13 0.525,1.4 | smd 1.45 x 0.35: 9 0.775,-0.5; 11 0.775,0.5 | smd 1.8 x 0.35: 10 0.6,0
61729-1011BLF = drill 0.92 square: 1 1.25,4.71 | drill 0.92: 2 -1.25,4.71; 3 -1.25,2.71; 4 1.25,2.71 | drill 2.3: SH1 -6.02,0; SH2 6.02,0

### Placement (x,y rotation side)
+3V3  43.13,66.36 0 top
+5V  26.49,63.09 180 top
AUDIO_JACK  92.58,6.97 270 top
BATTERIE1  5.06,64.63 90 top
BATTERIE2  5.06,72.25 90 top
BATTERYCHARGER  9.27,48.47 270 top
BOOT  67.65,75.45 180 top
BUZZER  46.7,46.76 0 top
C1  91.47,50.07 180 top
C2  56.05,71.39 0 top
C6  65.29,58.74 180 top
C7  15.07,70.14 270 top
C8  58.75,49.59 0 top
C9  57.51,46.41 270 top
C10  59.7,59.12 180 top
C11  59.7,52.77 180 top
C12  17.01,32.37 270 top
C13  77.36,55.88 0 top
C14  77.36,46.99 0 top
C15  80.33,11.14 0 top
C18  22.25,70.05 180 top
C19  22.25,65.28 180 top
C26  65.29,56.52 180 top
C_H-BRIDGE  27.42,20.3 0 top
CAUX  32.7,52.39 270 top
CIN  25.08,46.99 180 top
COUT  25.08,60.64 180 top
COUTX  25.08,58.42 180 top
D1  44.45,55.56 90 top
D2  18.91,33.01 90 top
D3  20.82,36.82 90 top
D4  20.82,39.04 90 top
D_H-BRIDGE1  21.79,25.58 0 top
D_H-BRIDGE2  19.17,22.73 0 top
DISPLAY  15,57.5 270 top
EXTENSIONS  97.59,68.07 90 bottom
GND  6.01,68.44 0 top
H-BRUECKE  15.44,14.15 180 top
IC2  29.24,67.51 270 top
JP1  83.19,5.4 270 top
L1  20.29,53.7 90 top
LED1  87,76.83 0 top
LED2  85.41,76.83 0 top
LED3  83.82,76.83 0 top
LED4  82.23,76.83 0 top
LED_CHARGE_GREEN  9.27,53.23 270 top
LED_CHARGE_RED  5.46,51.96 270 top
LED_INDICATOR  79.06,76.83 0 top
LED_LEFT  55.58,33.77 0 top
LED_MIDDLE  64.47,33.77 0 top
LED_RIGHT  73.36,33.77 0 top
LEFT  48.6,20.43 180 top
MOTOR  5.51,23.04 270 top
N-CHANNEL  12.44,52.28 0 top
NPN  47.41,55.53 0 top
ON/OFF  33.02,41.27 180 top
OPV  68.59,7.97 0 top
P-CHANNEL  5.66,59.39 90 top
POWER_LED  96.52,50.16 90 top
QUARTZ  62.88,47.69 90 top
QUARTZ2  60.98,55.94 90 top
R1  96.52,48.26 0 top
R2  60.18,71.39 180 top
R3  65.72,71.39 0 top
R4  69.85,71.39 0 top
R5  77.15,76.83 90 top
R6  12.12,48.15 270 top
R7  4.19,48.15 90 top
R8  6.41,48.15 90 top
R9  10.63,66.01 270 top
R10  12.85,66.01 90 top
R11  8.83,59.39 270 top
R12  59.73,46.41 90 top
R13  22.25,41.42 0 top
R14  78.42,64.14 0 top
R15  3.15,68.44 0 top
R16  74.62,11.14 0 top
R17  39.52,66.38 0 top
R18  66.99,2.22 180 top
R19  14.35,48.15 270 top
R20  12.85,70.14 90 top
R21  10.63,70.14 270 top
R22  78.42,66.67 0 top
R23  78.42,69.22 0 top
R24  78.42,71.75 0 top
R25  17.96,39.36 180 top
R26  17.96,37.13 180 top
R27  71.12,2.24 0 top
R28  50.42,55.38 270 top
R29  15.07,66.01 270 top
R30  55.39,29.32 180 top
R31  73.17,29.32 180 top
R32  64.27,29.32 180 top
R33  47.76,27.56 180 top
R34  42.1,55.7 90 top
R35  68.81,29.18 0 top
R36  49.76,29.82 0 top
R37  58.75,55.94 90 top
RENABLE  32.48,47.44 180 top
RESET  57.96,75.52 0 top
RFBB  32.93,58.28 90 top
RFBT  30.39,58.28 90 top
RIGHT  64.47,20.43 180 top
RPGOOD  35.47,59.87 90 top
SCHOTTKY1  7.76,56.22 0 top
SELECT  80.35,20.43 180 top
SIGNAL_IN  83.83,11.14 0 top
SIGNAL_OPAMP  73.98,1.94 0 top
ST_LINK  97.64,56.39 270 top
STM32  71.06,51.35 0 top
TRIMMER  77.16,5.43 180 top
U1  28.8,53.84 180 top
USB-B  9.2,36.82 270 top
VBAT  7.92,68.44 0 top
VBUS  22.09,33.33 0 top

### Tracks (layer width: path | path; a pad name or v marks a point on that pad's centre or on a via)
+3V3  (via drill 0.35)
  Top 0.254: STM32.36 76.41,55.27 C13.1 v74.82,55.88 | STM32.24 74.64,47.17 v74.82,46.99 C14.1 | C6.1 v66.24,60.33 | STM32.9 v68.58,50.1
  Top 0.305: BOOT.D BOOT.C | C26.1 C6.1 | STM32.48 67.32,56.52 C26.1 | STM32.1 66.24,54.73 C26.1 | ST_LINK.4 93.83,51.47 C1.1 94.23,48.26 R1.1 | OPV.4 65.6,7.97 64.78,8.79 64.78,14.34 69.8,19.36 72.67,19.36 SELECT.3
  Top 0.406: R2.2 59.23,68.76 | 59.23,68.76 56.83,66.36 | BOOT.D 63.18,75.86 63.18,70.52 61.42,68.76 59.23,68.76 | 56.83,66.36 v60.96,66.36 | R13.2 25.25,41.42 31.43,35.24 v41.59,35.24 | R17.2 43.11,66.38 +3V3.TP 56.83,66.36
  Bottom 0.305: v74.82,55.88 90.52,55.88 ST_LINK.4 | v74.82,46.99 73.56,45.73 73.56,24.42 72.67,23.53 72.67,19.36 SELECT.3
  Bottom 0.406: v60.96,66.36 63.18,66.36 68.26,61.28 68.26,60.01
  pour Bottom (no thermals): 65.44,45.54 79.41,45.54 79.41,61.29 65.44,61.29
  pour Bottom (isolate 0.305, no thermals): 40.67,15.05 85.63,15.05 85.63,36.05 40.67,36.05
  pour Bottom (no thermals): 89.22,57.78 100.01,57.78 100.01,46.67 89.22,46.67
+5V  (via drill 0.35)
  Top 0.305: RPGOOD.2 37.92,60.82 R34.2 | DISPLAY.2 17.14,60.91 17.14,62.87 17.78,63.5 21.87,63.5 C19.1
  Top 0.406: IC2.3 23.74,65.2 C19.1
  other vias: 27.62,56.52 27.62,57.78 27.62,59.05
  pour Bottom (no thermals): 28.57,61.91 25.72,61.91 25.72,55.24 28.57,55.24
  pour Top (isolate 0.254, no thermals): 28.57,55.24 25.4,55.24 25.4,63.82 22.86,63.82 22.86,66.36 27.62,66.36 27.62,62.23 36.2,62.23 36.2,60.33 31.43,60.33 31.43,58.42 28.57,58.42
BATTERY_LEVEL  (via drill 0.35)
  Top 0.254: v70.13,52.39 69.81,52.07 STM32.16 | v46.35,72.39 18.27,72.39 C7.2 16.15,68.11 16.15,66.14 R29.2
  Bottom 0.254: v70.13,52.39 70.31,52.57 70.31,60.31 58.22,72.39 v46.35,72.39
BOOT0  (via drill 0.35)
  Top 0.254: STM32.44 70.31,61.65 v69.47,62.49 | v66.67,69.22 R3.2
  Bottom 0.254: v69.47,62.49 66.67,65.29 v66.67,69.22
BUTTON_1
  Top 0.254: LEFT.1 42.35,25.3 44.61,27.56 R33.2 46.81,29.68 56.81,39.69 73.82,39.69 80.24,46.1 80.24,47.88 79.02,49.1 STM32.26
BUTTON_2
  Top 0.254: RIGHT.1 56.95,22.93 52.32,27.57 | 52.32,27.57 50.7,29.18 R36.2 | R36.2 | STM32.27 79.06,49.6 80.62,48.03 80.62,45.95 73.72,39.05 57.16,39.05 52.32,34.21 52.32,27.57
BUTTON_3
  Top 0.254: R35.2 69.75,27.27 SELECT.1 72.15,24.88 57.02,24.88 53.04,28.86 53.04,34.4 57.06,38.42 73.63,38.42 81,45.79 81,48.19 79.09,50.1 STM32.28
BUZZER
  Top 0.254: STM32.45 69.81,59.95 68.43,61.33 55.42,61.33 R28.1
CUSTOM1
  Top 0.254: STM32.38 73.31,63.18 74.26,64.14 R14.1
CUSTOM2
  Top 0.254: STM32.39 72.81,65.82 73.66,66.67 R22.1
CUSTOM3
  Top 0.254: R23.1 73.98,69.22 72.31,67.55 STM32.40
CUSTOM4
  Top 0.254: STM32.41 71.81,68.95 74.61,71.75 R24.1
DISPLAY_SCL  (via drill 0.35)
  Top 0.254: STM32.42 71.31,62.79 69.33,64.77 v40.32,64.77
  Bottom 0.254: DISPLAY.4 13.15,55.54 13.15,56.68 13.81,57.34 16.39,57.34 23.81,64.77 v40.32,64.77
DISPLAY_SDA  (via drill 0.35)
  Top 0.254: STM32.43 70.81,62.44 69.75,63.5 v40.32,63.5
  Bottom 0.254: DISPLAY.3 15.03,56.2 16.19,56.2 23.5,63.5 v40.32,63.5
GND  (via drill 0.3, 0.35, 0.5)  (1 unrouted)
  Top 0.254: RFBB.1 32.93,55.79 v32.38,55.24 31.73,54.59 U1.4
  Top 0.305: C10.1 v62.23,59.12 | C11.1 62.09,52.77 v62.32,52.54 | C9.1 56.15,47.36 v55.56,47.94 57.21,49.59 C8.1 | NPN.E v45.4,54.43
  Top 0.406: R11.1 9.8,61.31 DISPLAY.1 | BATTERIE2.1 6.99,71.59 6.99,69.42 GND.TP
  Bottom 0.305: v45.4,54.43 53.03,54.43 53.75,55.15
  Bottom 0.406: 1.27,45.09 2.86,43.5 v4.76,43.5 | 1.27,55.24 3.17,53.34 v4.13,53.34 | 17.46,69.53 19.05,67.94 v20.32,67.94 | 1.27,46.99 2.22,46.04 v9.21,46.04 | 42.86,73.52 53.75,62.63 53.75,61.18 | 53.75,61.18 53.75,59.28 | 53.75,59.28 53.75,55.15 53.75,50.7 | v55.56,47.94 55.56,48.9 53.75,50.7 | 1.27,29.53 2.86,27.94 v50.8,27.94 | 13.02,73.52 14.74,73.52 v15.56,72.71 | v75.56,44.77 75.56,34.42 75.75,34.23 75.75,13.5 77.16,12.1 TRIMMER.2 | 53.75,59.28 57.15,55.88 | v66.36,47.31 64.14,45.09 54.93,45.09 53.75,46.26 53.75,50.7 | v63.82,60.33 54.61,60.33 53.75,61.18
  Bottom 0.508: v2.86,26.35 1.27,27.94 1.27,29.53 1.27,45.09 1.27,46.99 1.27,55.24 1.27,69.73 BATTERIE2.1 13.02,73.52 16.65,73.52 | 16.65,73.52 17.46,72.71 17.46,69.53 17.46,64.77 | 16.65,73.52 42.86,73.52 52.56,73.52 v54.61,75.56 | 17.46,64.77 17.46,63.5 | DISPLAY.1 15.27,61.31 17.46,63.5 | 17.46,64.77 16.19,63.5 v14.92,63.5 | 17.46,63.5 17.46,62.55 v18.73,61.28
  other vias: 34.41,53.86 21.91,60.64 21.59,46.67 23.5,48.58 22.86,58.42 29.21,53.27 29.2,54.42 34.41,50.36 34.41,52.11 21.59,48.26 21.59,59.05
  pour Top (isolate 0.305, no thermals): 30.5,27.5 0.5,27.5 0.5,17.5 30.5,17.5
  pour Top (isolate 0.305, no thermals): 25.14,29.23 3.92,29.23 3.92,44.55 25.14,44.55
  pour Top (isolate 0.305, no thermals): 16.34,63.15 9.36,63.15 9.36,73 16.34,73
  pour Top (isolate 0.305, no thermals): 10.03,61.28 10.03,55.15 3.4,55.15 3.4,61.28
  pour Bottom (isolate 0.305, no thermals): 64.78,50.86 54.94,50.86 54.94,44.19 64.78,44.19
  pour Bottom (isolate 0.305, no thermals): 56.53,60.38 56.53,51.49 62.88,51.49 62.88,60.38
  pour Top (isolate 0.305, no thermals): 99.5,0.5 64.55,0.5 64.55,12.82 99.5,12.82
  pour Top (no thermals): 79.91,43.77 63.06,43.77 63.06,61.48 79.91,61.48
  pour Top (isolate 0.305, no thermals): 40.17,14.55 86.13,14.55 86.13,36.55 40.17,36.55
  pour Top (isolate 0.305, no thermals): 3.55,45.61 14.98,45.61 14.98,53.87 3.55,53.87
  pour Top (isolate 0.305, no thermals): 53.98,79.69 100.01,79.69 100.01,46.67 89.22,46.67 89.22,74.61 72.71,74.61 72.71,68.58 53.98,68.58
  pour Top (isolate 0.203, rank 2, no thermals): 24.77,45.72 24.77,53.66 28.57,53.66 28.57,53.98 24.77,53.98 24.77,62.23 17.78,62.23 17.78,45.72
  pour Bottom (rank 2, no thermals): 36.51,45.4 36.51,62.55 17.46,62.55 17.46,45.4
  pour Top (isolate 0.127, no thermals): 29.53,52.78 29.53,54.61 29.21,54.61 29.21,55.56 28.89,55.56 28.89,53.02 29.29,53.02 29.29,52.07 29.77,52.07 29.77,52.78
  pour Top (isolate 0.254, no thermals): 32.07,52.07 32.07,49.53 35.56,49.53 35.56,54.61 33.34,54.61 33.34,52.07
  pour Top (no thermals): 19.05,71.44 19.05,63.82 21.59,63.82 21.59,66.99 27.3,66.99 27.3,71.44
L1  (via drill 0.3, 0.35)
  other vias: 23.18,52.7 23.18,51.44 22.23,50.8 20.95,50.8 26.63,53.14
  pour Bottom (no thermals): 28.57,53.02 28.57,53.58 18.1,53.58 18.1,50.16 25.08,50.16 25.08,53.02
  pour Top (isolate 0.254, no thermals): 24.13,49.85 18.1,49.85 18.1,53.34 24.13,53.34
  pour Top (isolate 0.127, no thermals): 28.57,53.02 28.57,53.34 26.35,53.34 26.35,53.02
L2  (via drill 0.3, 0.35)
  other vias: 23.18,54.61 23.18,55.88 21.91,56.52 20.64,56.52 26.63,54.49
  pour Bottom (no thermals): 28.57,54.05 18.1,54.05 18.1,57.15 25.08,57.15 25.08,54.61 28.57,54.61
  pour Top (isolate 0.254, no thermals): 24.13,53.98 18.1,53.98 18.1,57.47 24.13,57.47
  pour Top (isolate 0.127, no thermals): 28.57,54.29 28.57,54.61 26.35,54.61 26.35,54.29
LED_LEFT
  Top 0.254: LED_LEFT.A 56.85,35.35 59.28,37.78 73.53,37.78 81.51,45.76 81.51,48.22 79.13,50.6 STM32.29
LED_MIDDLE
  Top 0.254: STM32.30 79.17,51.1 82.08,48.19 82.08,45.47 73.86,37.26 69.23,37.26 LED_MIDDLE.A
LED_RIGHT
  Top 0.254: STM32.31 79.21,51.6 82.46,48.35 82.46,41.59 LED_RIGHT.A
MOTOR_PWM1
  Top 0.254: STM32.18 70.81,41.59 70.17,40.96 55.77,40.96 40.71,25.9 27.18,25.9 D_H-BRIDGE1.A
MOTOR_PWM2
  Top 0.254: D_H-BRIDGE2.A 39.12,22.73 56.72,40.32 70.08,40.32 71.31,41.55 STM32.19
MOTORA
  Top 0.406: MOTOR.2 8.03,26.82 17.22,26.82 17.98,26.07 H-BRUECKE.2
MOTORB
  Top 0.406: MOTOR.1 12.07,21.77 12.89,20.94 H-BRUECKE.6
N$1
  Top 0.305: POWER_LED.A 97.57,48.36 R1.2
N$2
  Top 0.305: R5.1 78.96,75.89 LED_INDICATOR.A
N$3
  Top 0.406: P-CHANNEL.3 4.76,59.19 4.76,57.15 5.7,56.22 SCHOTTKY1.C 7.95,54.93 16.17,54.93 16.93,54.17 16.93,45.5 18.61,43.81 27.94,43.81 ON/OFF.3
N$4
  Top 0.508: R9.2 R10.1
N$5
  Top 0.305: R3.1 64.65,71.52 BOOT.B BOOT.A 70.65,71.54 R4.2
N$6
  Top 0.406: H-BRUECKE.3 D_H-BRIDGE1.C
N$7
  Top 0.305: R18.1 67.95,2.23 R27.1 71.06,3.13 OPV.8
N$8
  Top 0.508: BATTERYCHARGER.5 10.25,47.2 R6.2 R19.2
N$9
  Top 0.508: R8.2 6.51,49.2 LED_CHARGE_RED.C 8.95,51.96 10.22,50.69 | 10.22,50.69 BATTERYCHARGER.1 | N-CHANNEL.1 10.71,51.18 10.22,50.69
N$11
  Top 0.508: LED_CHARGE_GREEN.A 5.68,53.23 LED_CHARGE_RED.A 4.41,49.32 R7.2
N$12
  Top 0.508: LED_CHARGE_GREEN.C 10.46,53.38 N-CHANNEL.3
N$13
  Top 0.406: IC2.4 28.92,67.51 27.91,68.52 24.48,68.52 23.65,69.34 C18.1
  pour Top (isolate 0.305, no thermals): 31.14,69.73 31.14,65.28 32.73,63.7 39.08,63.7 39.08,71.32 32.73,71.32
N$14
  Top 0.406: D_H-BRIDGE2.C 14.16,22.65 H-BRUECKE.5
N$16
  Top 0.305: TRIMMER.3 OPV.9 71.57,5.43 72.4,4.61 72.4,2.56 R27.2
N$19
  Top 0.305: R30.2 54.31,29.45 LED_LEFT.C
N$20
  Top 0.305: R31.2 72.09,29.45 LED_RIGHT.C
N$23
  Top 0.305: R32.2 63.2,29.44 LED_MIDDLE.C
N$29
  Top 0.305: USB-B.3 13.2,39.36 R25.2
N$30
  Top 0.305: USB-B.2 16.07,38.07 R26.2
N$39
  Top 0.305: EXTENSIONS.1 93.65,64.14 85.72,64.14 | 85.72,64.14 R14.2 | LED1.A 87,65.41 85.72,64.14
N$46
  Top 0.508: R21.1 R20.2
N$47
  Top 0.508: R20.1 R10.2 R29.1
N$48  (via drill 0.35)
  Top 0.305: R22.2 83.19,66.67 | 83.19,66.67 85.41,68.9 LED2.A | 83.19,66.67 v85.72,66.67
  Bottom 0.305: v85.72,66.67 93.65,66.67 EXTENSIONS.2
N$49  (via drill 0.35)
  Top 0.305: R23.2 82.55,69.22 | 82.55,69.22 83.82,70.48 LED3.A | 82.55,69.22 v84.14,69.22
  Bottom 0.305: v84.14,69.22 93.65,69.22 EXTENSIONS.3
N$50  (via drill 0.35)
  Top 0.305: R24.2 80.64,71.75 | 80.64,71.75 82.23,73.34 LED4.A | 80.64,71.75 v82.87,71.75
  Bottom 0.305: v82.87,71.75 93.65,71.75 EXTENSIONS.4
N$51
  Top 0.406: BATTERIE2.2 4.67,70.98 2.21,68.51 R15.1
N$52
  Top 0.305: C15.1 R16.2 75.57,9.74 72.53,6.7 OPV.10
N$53
  Top 0.406: BATTERIE1.1 5.06,67.49 R15.2
N$54
  Top 0.305: BUZZER.+ 47.41,48.34 NPN.C 47.38,56.66 D1.A
N$55
  Top 0.305: R34.1 42.38,54.46 D1.C 44.45,46.79 BUZZER.-
N$56
  Top 0.305: R28.2 NPN.B
N$60
  Top 0.254: CAUX.1 32.7,53.66 32.27,54.09 U1.3
N$61
  Top 0.254: U1.2 30.86,53.59 31.75,52.7 31.75,49.41 32.27,48.9 35.56,48.9 36.06,49.39 36.06,58.34 RPGOOD.1
N$62
  Top 0.254: U1.5 29.53,56.16 30.39,57.02 RFBT.1 31.03,57.34 RFBB.2
N$64
  Top 0.203: U1.14 29.03,52.07
  Top 0.254: RENABLE.2 29.84,47.44 29.12,48.17 29.03,48.26 29.03,52.07
OSC32IN
  Top 0.254: C10.2 R37.2 59.05,57.19 QUARTZ2.2 61.8,57.19 65.9,53.1 STM32.3
OSC32OUT
  Top 0.254: C11.2 R37.1 60.67,54.99 QUARTZ2.1 61.24,54.69 63.34,52.6 STM32.4
OSCIN
  Top 0.254: R12.2 59.73,49.56 C8.2 62.78,49.59 QUARTZ.2 65.29,52.1 STM32.5
OSCOUT
  Top 0.254: C9.2 R12.1 62.65,45.46 QUARTZ.1 65.04,47.85 65.04,50.6 66.04,51.6 STM32.6
PAD  (via drill 1)
  other vias: 23.43,8.01 3.44,12.01 7.43,12.01 3.44,8.01 7.43,8.01 7.43,4.01 11.44,8.01 23.43,12.01 27.43,12.01 27.43,8.01 19.43,8.01 15.44,8.01 15.44,4.01 11.44,4.01 19.43,4.01 23.43,4.01 27.43,4.01
  pour Top (isolate 0.305, no thermals): 0.5,0.5 30.5,0.5 30.5,17 0.5,17
PC13  (via drill 0.35)
  Top 0.254: v75.25,77.47 75.56,77.78 R5.2 | STM32.2 v71.44,53.6
  Bottom 0.254: v75.25,77.47 74.3,76.52 74.3,69.85 71.44,66.99 v71.44,53.6
RESET  (via drill 0.35)
  Top 0.254: STM32.7 67.94,51.1 68.58,51.73 v68.58,52.02 | C2.1 55.1,70.32 55.88,69.54 v55.88,69.53 | 61.13,73.47 R2.1
  Top 0.305: C2.1 54.96,71.53 RESET.C RESET.D 61.13,73.47
  Bottom 0.254: v68.58,52.02 68.58,56.85 55.89,69.53 v55.88,69.53
SIGNAL_IN
  Top 0.305: SIGNAL_IN.TP C15.2 81.28,7.3 JP1.2
SIGNAL_IN_1
  Top 0.305: JP1.1 90.14,7.94 AUDIO_JACK.5
SIGNAL_IN_2
  Top 0.305: AUDIO_JACK.2 88.99,2.86 JP1.3
SIGNAL_OPAMP  (via drill 0.35)
  Top 0.254: SIGNAL_OPAMP.TP 73.64,1.94 72.84,1.15 67.12,1.15 R18.2
  Top 0.305: v67.31,44.45 67.14,44.62 67.14,48.6 STM32.12 | v67.94,16.19 67.94,4.12 R18.2
  Bottom 0.305: v67.94,16.19 67.94,43.81 v67.31,44.45
SWDCLK
  Top 0.254: STM32.37 73.81,56.2 74.95,57.34 93.51,57.34 ST_LINK.2
SWDIO
  Top 0.254: STM32.34 79.58,53.1 81.28,54.8 93.51,54.8 ST_LINK.3
USB+  (via drill 0.35)
  Top 0.254: D4.2 v22.23,39.39 | STM32.33 72.8,52.6 v71.96,51.75
  Top 0.305: 18.94,39.39 D4.2 20.82,41.42 R13.1
  Top 0.406: R25.1 18.94,39.39
  Bottom 0.254: v71.96,51.75 59.28,39.07 22.54,39.07 v22.23,39.39
USB-  (via drill 0.35)
  Top 0.254: D3.2 v22.23,37.17 | v73.23,51.75 73.57,52.1 STM32.32
  Top 0.305: 18.94,37.17 D3.2
  Top 0.406: R26.1 18.94,37.17
  Bottom 0.254: v73.23,51.75 58.33,36.85 22.54,36.85 v22.23,37.17
VBAT  (via drill 0.35)
  Top 0.406: C_H-BRIDGE.+ 19.26,20.3 H-BRUECKE.1 | P-CHANNEL.2 6.76,61.61 5.06,63.31 BATTERIE1.2 7.92,66.22 VBAT.TP 8.66,69.19 R21.2 | BATTERYCHARGER.3 v8.32,51.07 | v2.86,51.07 1.91,52.03 1.91,52.39
  Top 0.508: 19.26,20.3 19.26,20.24 19.97,19.53 19.97,18.27 19.77,18.07 11.1,18.07 10.9,18.27 10.9,19.53 11.62,20.26 H-BRUECKE.7 10.48,20.32 4.13,20.32 1.91,22.54 1.91,52.39 1.91,61.45 3.76,63.31 5.06,63.31
  Bottom 0.406: v8.32,51.07 v2.86,51.07
VBUS  (via drill 0.35)
  Top 0.305: 17.01,33.35 C12.1 | BATTERYCHARGER.4 | 6.41,47.17 R8.1 | D2.2 22.05,33.36 VBUS.TP
  Top 0.406: C12.1 16.98,33.35 16.13,33.35 USB-B.1 12.79,34.45 11.45,34.45 6.41,39.49 R8.1 | D2.2 18.9,33.35 17.01,33.35 | SCHOTTKY1.A 8.86,58.41 | P-CHANNEL.1 R11.2 8.86,58.41 | v11.43,58.1 11.11,58.42 8.87,58.42 8.86,58.41
  Top 0.508: R7.1 4.22,47.17 6.41,47.17 | R8.1 8.28,47.2 BATTERYCHARGER.4
  Bottom 0.406: v11.43,58.1 11.43,39.69 10.79,39.05 10.79,35.11 11.45,34.45 12.79,34.45 USB-B.1
VIN  (via drill 0.35, 0.5)
  Top 0.254: U1.1 30.48,53.09 30.8,52.77 v30.8,51.12
  Top 0.406: ON/OFF.2 33.02,45.09 v35.24,47.31
  Bottom 0.254: v27.62,51.12 v30.8,51.12
  other vias: 27.62,48.58 27.62,49.85
  pour Bottom (no thermals): 28.57,52.39 25.72,52.39 25.72,45.72 28.57,45.72
  pour Top (isolate 0.254, no thermals): 28.57,52.7 25.4,52.7 25.4,45.72 36.2,45.72 36.2,48.58 32.38,48.58 32.38,46.35 28.57,46.35
(copper drawn outside any net)
  shapes: Top area x2980

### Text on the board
Top: AutoTuner V3 - Maturaprojekt / Gabriel Unterweger - 5BEL / TFO Meran 23 / 24
tStop: AutoTuner V3 - Maturaprojekt / Gabriel Unterweger - 5BEL / TFO Meran 23 / 24
Einteilung: Reset | Boot | BuildInLED | + - | Battery 1 | Extenions | GND | VBAT | +3V3 | +5V | 5V->3V3 | + - | VBAT LVL | Battery 2 | ST-Link | V Selection | Power | BAT Charger | microcontroller | Buzzer | VBUS | USB | MOTOR | DC Driver | Buttons / LEDs | SIGNAL_IN | SIGNAL_OPAMP | Input

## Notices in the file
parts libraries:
crystal-geyer_V1_0: Copyright: Geyer-Electronic
SparkFun-Switches: Licensing: Creative Commons ShareAlike 4.0 International - https://creativecommons.org/licenses/by-sa/4.0
